FUNCTION "FC_GRP_82" : VOID
TITLE =GROUP =82
{ S7_language := '9(1) Angielski (Stany Zjednoczone)  11.01.2022  09:45:15' }
VERSION : 0.1


VAR_TEMP
  CL : "UDT_CABINET";	//CABINET LOCAL
  CR : "UDT_CABINET";	//CABINET REMOTE
  RelError : BOOL ;	//ERROR RELEASE
  RelErrorCL : BOOL ;	//ERROR RELEASE FROM CABINET LOCAL
  RelErrorCR : BOOL ;	//ERROR RELEASE FROM CABINET REMOTE
  RelControl : BOOL ;	//CONTROL RELEASE
  RelControlCL : BOOL ;	//CONTROL RELEASE FROM CABINET LOCAL
  RelControlCR : BOOL ;	//CONTROL RELEASE FROM CABINET REMOTE
  ErrorConfirm : BOOL ;	//ERROR CONFIRM
  AutoOn : BOOL ;	//AUTOMATIC ON
  AutoOff : BOOL ;	//AUTOMATIC OFF
  LAMP_ON : BOOL ;
  Setpoint_82FAN91_reached : BOOL ;
  Setpoint_82FAN91_div : BOOL ;
  Setpoint_82FAN92_reached : BOOL ;
  Setpoint_82FAN92_div : BOOL ;
END_VAR
BEGIN
NETWORK
TITLE =GLOBAL SIGNALS
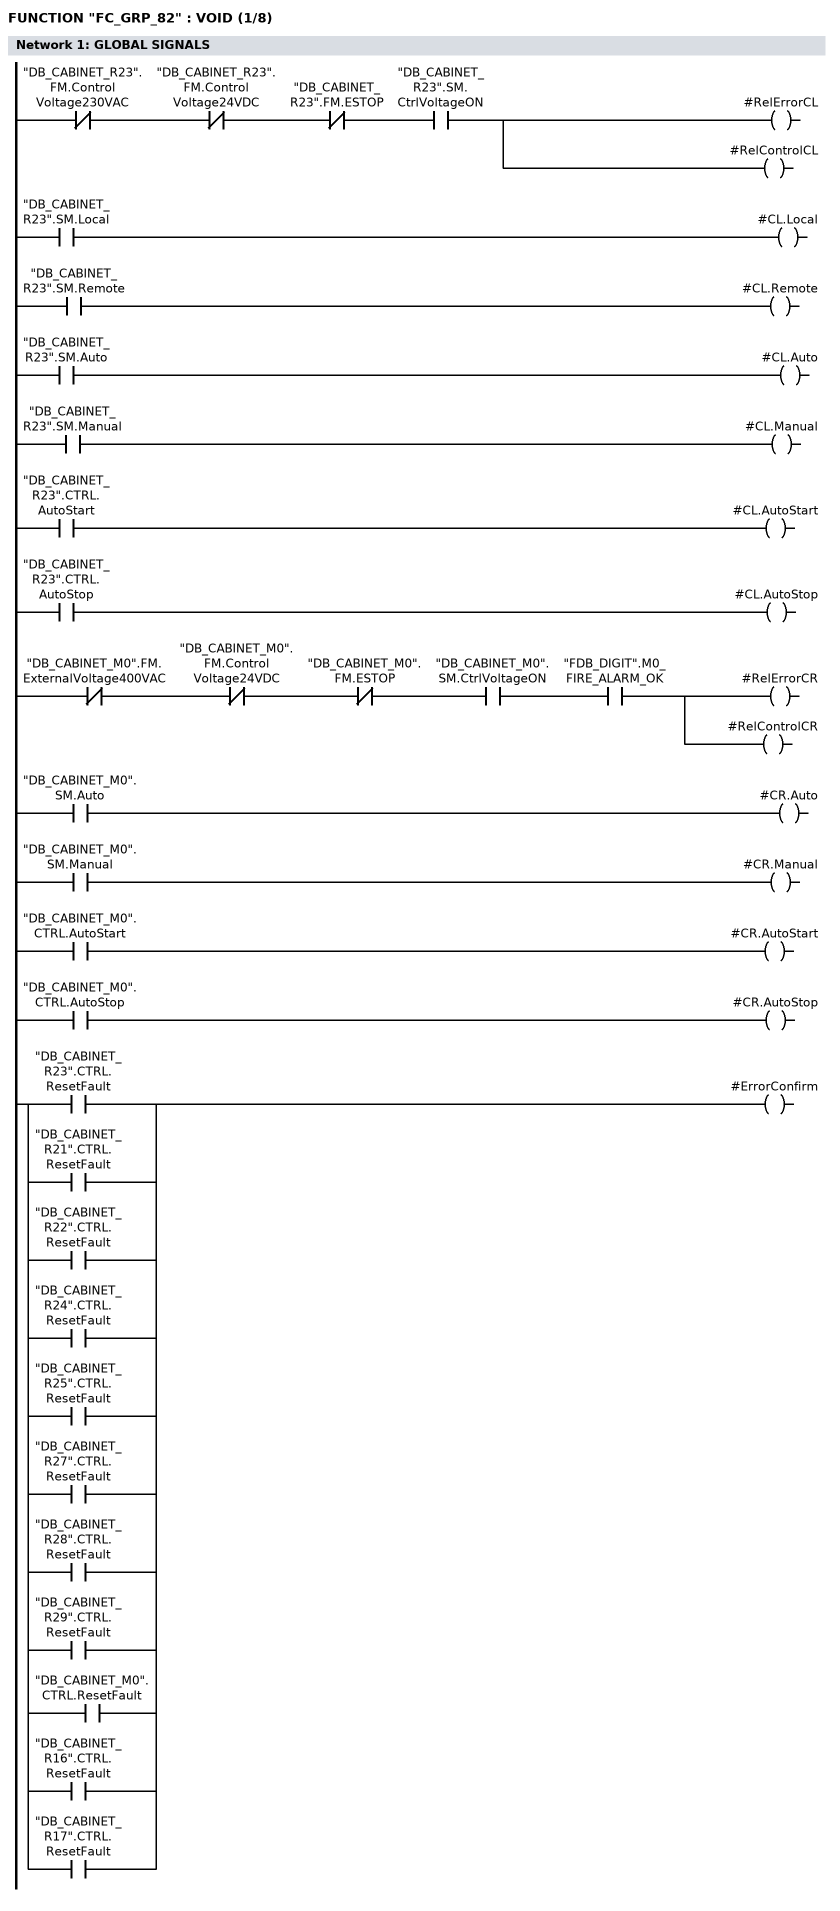
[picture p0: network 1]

// LOCAL
      UN    "DB_CABINET_R23".FM.ControlVoltage230VAC;
      UN    "DB_CABINET_R23".FM.ControlVoltage24VDC;
//      UN    "DB_CABINET_R23".FM.ControlVoltage230VAC_MS
      UN    "DB_CABINET_R23".FM.ESTOP;
      U     "DB_CABINET_R23".SM.CtrlVoltageON;
      =     #RelErrorCL;
      =     #RelControlCL;

      U     "DB_CABINET_R23".SM.Local;
      =     #CL.Local;
      U     "DB_CABINET_R23".SM.Remote;
      =     #CL.Remote;
      U     "DB_CABINET_R23".SM.Auto;
      =     #CL.Auto;
      U     "DB_CABINET_R23".SM.Manual;
      =     #CL.Manual;
      U     "DB_CABINET_R23".CTRL.AutoStart;
      =     #CL.AutoStart;
      U     "DB_CABINET_R23".CTRL.AutoStop;
      =     #CL.AutoStop;

// REMOTE
      UN    "DB_CABINET_M0".FM.ExternalVoltage400VAC;
      UN    "DB_CABINET_M0".FM.ControlVoltage24VDC;
//      UN    "DB_CABINET_M0".FM.ControlVoltage230VAC_MS
      UN    "DB_CABINET_M0".FM.ESTOP;
      U     "DB_CABINET_M0".SM.CtrlVoltageON;
      U     "FDB_DIGIT".M0_FIRE_ALARM_OK;
      =     #RelErrorCR;
      =     #RelControlCR;

      U     "DB_CABINET_M0".SM.Auto;
      =     #CR.Auto;
      U     "DB_CABINET_M0".SM.Manual;
      =     #CR.Manual;
      U     "DB_CABINET_M0".CTRL.AutoStart;
      =     #CR.AutoStart;
      U     "DB_CABINET_M0".CTRL.AutoStop;
      =     #CR.AutoStop;

      U     "DB_CABINET_R23".CTRL.ResetFault;
      O     "DB_CABINET_R21".CTRL.ResetFault;
      O     "DB_CABINET_R22".CTRL.ResetFault;
      O     "DB_CABINET_R24".CTRL.ResetFault;
      O     "DB_CABINET_R25".CTRL.ResetFault;
      O     "DB_CABINET_R27".CTRL.ResetFault;
      O     "DB_CABINET_R28".CTRL.ResetFault;
      O     "DB_CABINET_R29".CTRL.ResetFault;
      O     "DB_CABINET_M0".CTRL.ResetFault;
      O     "DB_CABINET_R16".CTRL.ResetFault;
      O     "DB_CABINET_R17".CTRL.ResetFault;
      =     #ErrorConfirm;

NETWORK
TITLE ==82FTR20-B33 FILTER PRESSURE MONITORING
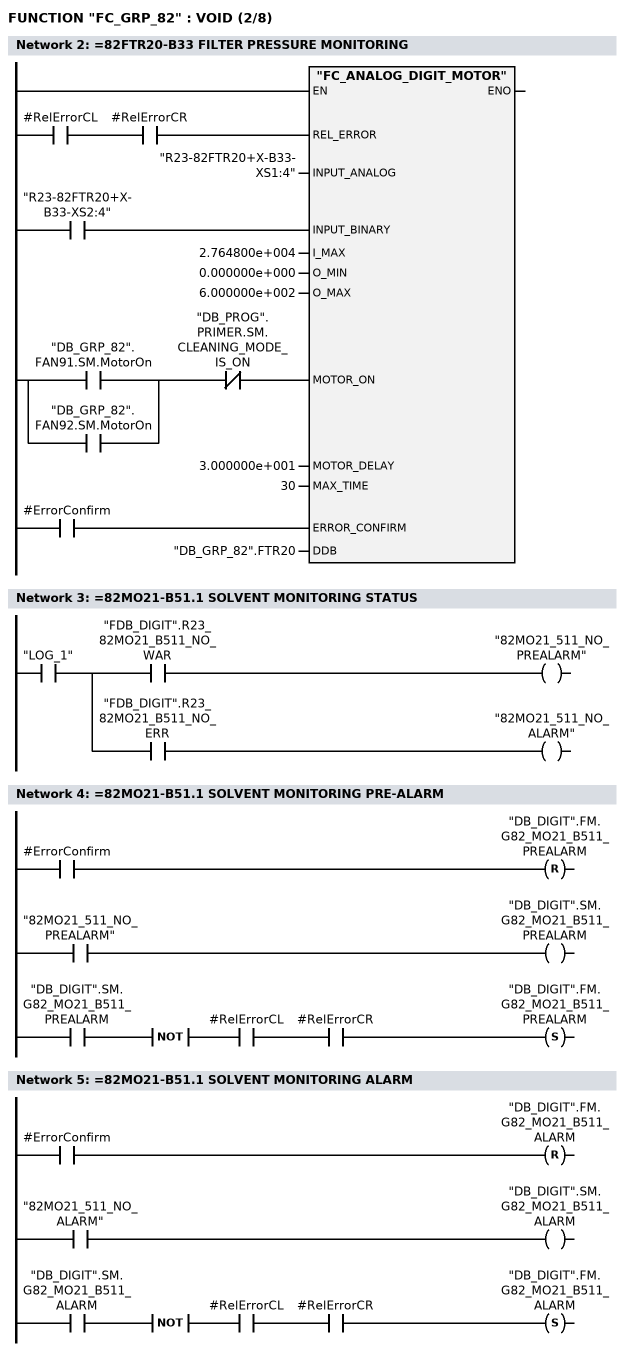
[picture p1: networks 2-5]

      U     #RelErrorCL;
      U     #RelErrorCR;
      =     L      6.0;
      BLD   103;
      U     "R23-82FTR20+X-B33-XS2:4";
      =     L      6.1;
      BLD   103;
      U(    ;
      O     "DB_GRP_82".FAN91.SM.MotorOn;
      O     "DB_GRP_82".FAN92.SM.MotorOn;
      )     ;
      UN    "DB_PROG".PRIMER.SM.CLEANING_MODE_IS_ON;
      =     L      6.2;
      BLD   103;
      U     #ErrorConfirm;
      =     L      6.3;
      BLD   103;
      CALL "FC_ANALOG_DIGIT_MOTOR" (
           REL_ERROR                := L      6.0,
           INPUT_ANALOG             := "R23-82FTR20+X-B33-XS1:4",
           INPUT_BINARY             := L      6.1,
           I_MAX                    := 2.764800e+004,
           O_MIN                    := 0.000000e+000,
           O_MAX                    := 6.000000e+002,
           MOTOR_ON                 := L      6.2,
           MOTOR_DELAY              := 3.000000e+001,
           MAX_TIME                 := 30,
           ERROR_CONFIRM            := L      6.3,
           DDB                      := "DB_GRP_82".FTR20);
      NOP   0;
NETWORK
TITLE ==82MO21-B51.1 SOLVENT MONITORING STATUS

      U     "LOG_1";
      =     L      6.0;
      U     L      6.0;
      U     "FDB_DIGIT".R23_82MO21_B511_NO_WAR;
      =     "82MO21_511_NO_PREALARM";
      U     L      6.0;
      U     "FDB_DIGIT".R23_82MO21_B511_NO_ERR;
      =     "82MO21_511_NO_ALARM";
NETWORK
TITLE ==82MO21-B51.1 SOLVENT MONITORING PRE-ALARM

      U     #ErrorConfirm;
      R     "DB_DIGIT".FM.G82_MO21_B511_PREALARM;
      U     "82MO21_511_NO_PREALARM";
      =     "DB_DIGIT".SM.G82_MO21_B511_PREALARM;
      U     "DB_DIGIT".SM.G82_MO21_B511_PREALARM;
      NOT   ;
      U     #RelErrorCL;
      U     #RelErrorCR;
      S     "DB_DIGIT".FM.G82_MO21_B511_PREALARM;
      NOP   0;
NETWORK
TITLE ==82MO21-B51.1 SOLVENT MONITORING ALARM

      U     #ErrorConfirm;
      R     "DB_DIGIT".FM.G82_MO21_B511_ALARM;
      U     "82MO21_511_NO_ALARM";
      =     "DB_DIGIT".SM.G82_MO21_B511_ALARM;
      U     "DB_DIGIT".SM.G82_MO21_B511_ALARM;
      NOT   ;
      U     #RelErrorCL;
      U     #RelErrorCR;
      S     "DB_DIGIT".FM.G82_MO21_B511_ALARM;
      NOP   0;
NETWORK
TITLE ==82MO21-B51.1 SOLVENT MONITORING ANALOG
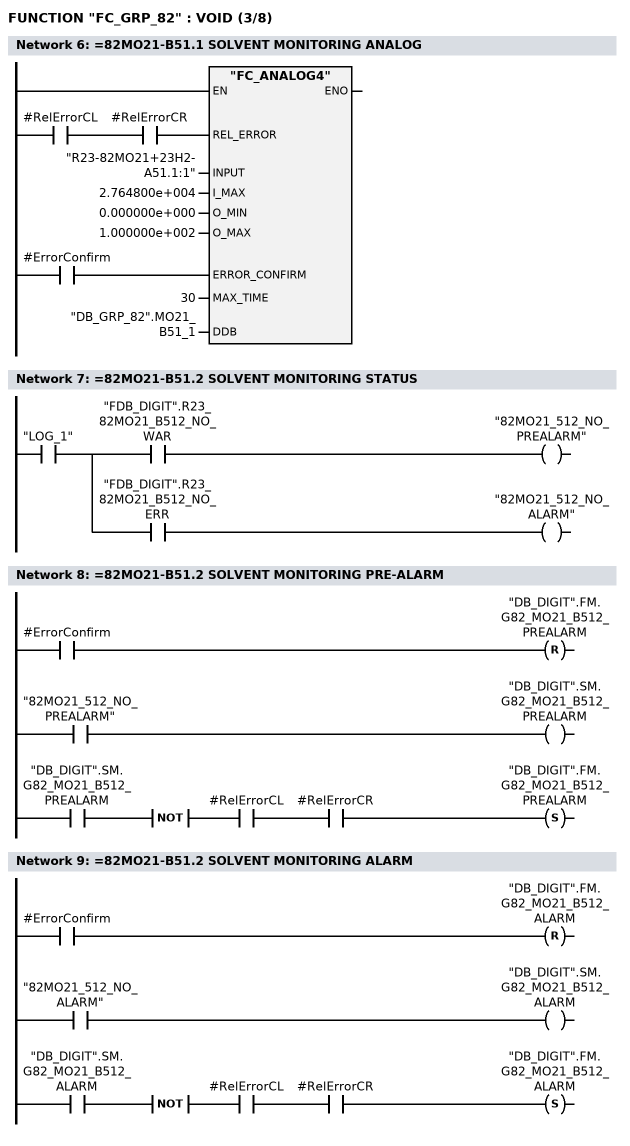
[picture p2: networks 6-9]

      U     #RelErrorCL;
      U     #RelErrorCR;
      =     L      6.0;
      BLD   103;
      U     #ErrorConfirm;
      =     L      6.1;
      BLD   103;
      CALL "FC_ANALOG4" (
           REL_ERROR                := L      6.0,
           INPUT                    := "R23-82MO21+23H2-A51.1:1",
           I_MAX                    := 2.764800e+004,
           O_MIN                    := 0.000000e+000,
           O_MAX                    := 1.000000e+002,
           ERROR_CONFIRM            := L      6.1,
           MAX_TIME                 := 30,
           DDB                      := "DB_GRP_82".MO21_B51_1);
      NOP   0;
NETWORK
TITLE ==82MO21-B51.2 SOLVENT MONITORING STATUS

      U     "LOG_1";
      =     L      6.0;
      U     L      6.0;
      U     "FDB_DIGIT".R23_82MO21_B512_NO_WAR;
      =     "82MO21_512_NO_PREALARM";
      U     L      6.0;
      U     "FDB_DIGIT".R23_82MO21_B512_NO_ERR;
      =     "82MO21_512_NO_ALARM";
NETWORK
TITLE ==82MO21-B51.2 SOLVENT MONITORING PRE-ALARM

      U     #ErrorConfirm;
      R     "DB_DIGIT".FM.G82_MO21_B512_PREALARM;
      U     "82MO21_512_NO_PREALARM";
      =     "DB_DIGIT".SM.G82_MO21_B512_PREALARM;
      U     "DB_DIGIT".SM.G82_MO21_B512_PREALARM;
      NOT   ;
      U     #RelErrorCL;
      U     #RelErrorCR;
      S     "DB_DIGIT".FM.G82_MO21_B512_PREALARM;
      NOP   0;
NETWORK
TITLE ==82MO21-B51.2 SOLVENT MONITORING ALARM

      U     #ErrorConfirm;
      R     "DB_DIGIT".FM.G82_MO21_B512_ALARM;
      U     "82MO21_512_NO_ALARM";
      =     "DB_DIGIT".SM.G82_MO21_B512_ALARM;
      U     "DB_DIGIT".SM.G82_MO21_B512_ALARM;
      NOT   ;
      U     #RelErrorCL;
      U     #RelErrorCR;
      S     "DB_DIGIT".FM.G82_MO21_B512_ALARM;
      NOP   0;
NETWORK
TITLE ==82MO21-B51.2 SOLVENT MONITORING ANALOG
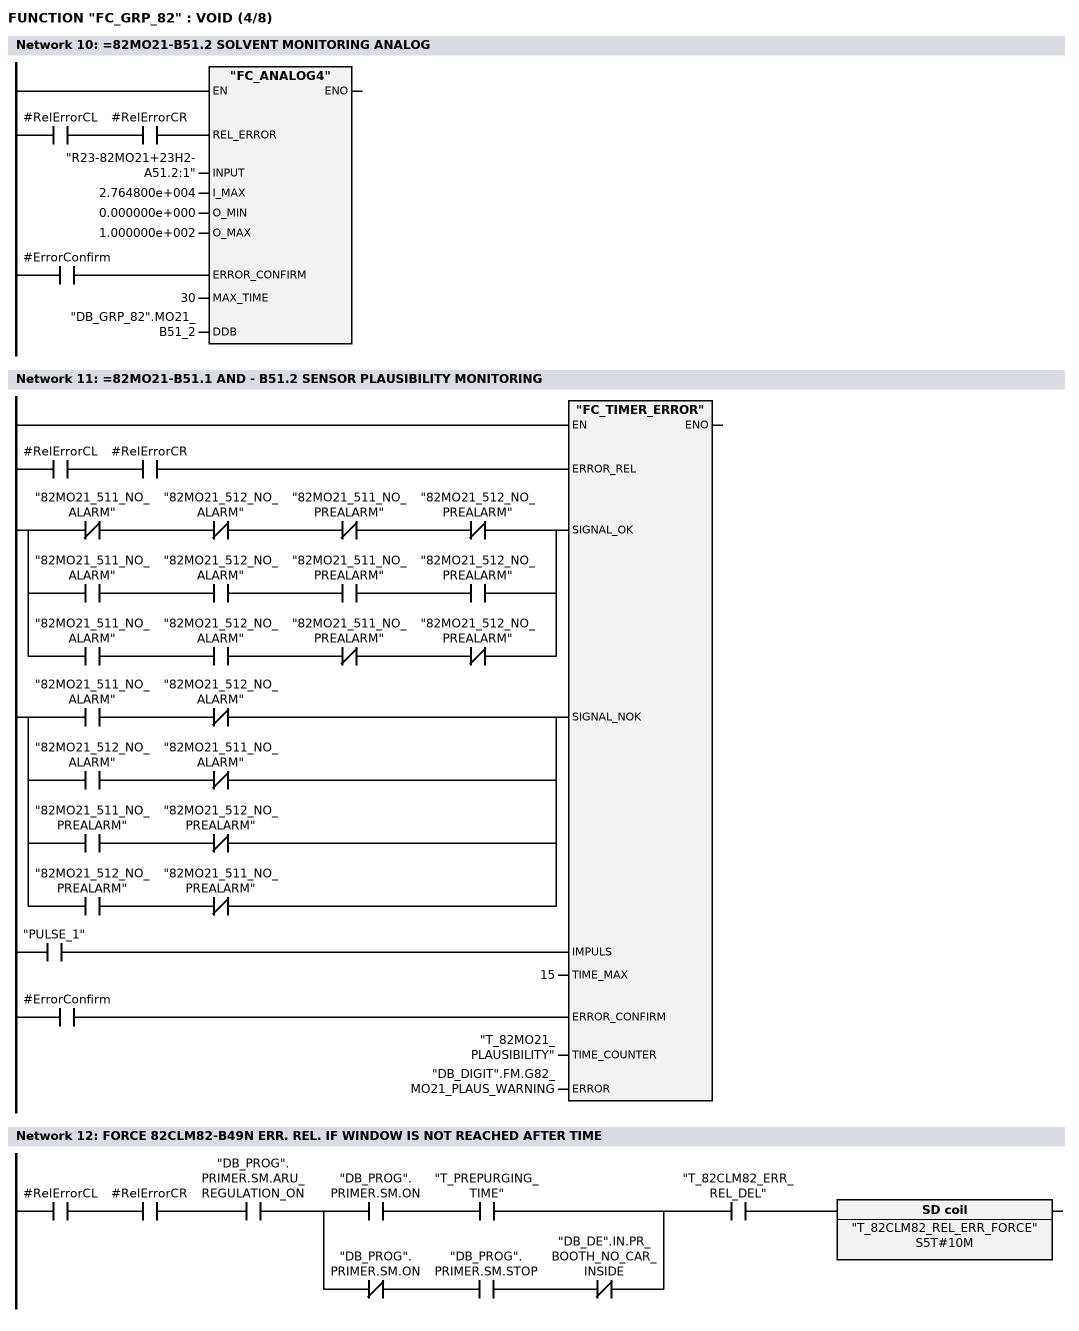
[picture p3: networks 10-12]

      U     #RelErrorCL;
      U     #RelErrorCR;
      =     L      6.0;
      BLD   103;
      U     #ErrorConfirm;
      =     L      6.1;
      BLD   103;
      CALL "FC_ANALOG4" (
           REL_ERROR                := L      6.0,
           INPUT                    := "R23-82MO21+23H2-A51.2:1",
           I_MAX                    := 2.764800e+004,
           O_MIN                    := 0.000000e+000,
           O_MAX                    := 1.000000e+002,
           ERROR_CONFIRM            := L      6.1,
           MAX_TIME                 := 30,
           DDB                      := "DB_GRP_82".MO21_B51_2);
      NOP   0;
NETWORK
TITLE ==82MO21-B51.1 AND - B51.2 SENSOR PLAUSIBILITY MONITORING

      U     #RelErrorCL;
      U     #RelErrorCR;
      =     L      6.0;
      BLD   103;
      U(    ;
      UN    "82MO21_511_NO_ALARM";
      UN    "82MO21_512_NO_ALARM";
      UN    "82MO21_511_NO_PREALARM";
      UN    "82MO21_512_NO_PREALARM";
      O     ;
      U     "82MO21_511_NO_ALARM";
      U     "82MO21_512_NO_ALARM";
      U     "82MO21_511_NO_PREALARM";
      U     "82MO21_512_NO_PREALARM";
      O     ;
      U     "82MO21_511_NO_ALARM";
      U     "82MO21_512_NO_ALARM";
      UN    "82MO21_511_NO_PREALARM";
      UN    "82MO21_512_NO_PREALARM";
      )     ;
      =     L      6.1;
      BLD   103;
      U(    ;
      U     "82MO21_511_NO_ALARM";
      UN    "82MO21_512_NO_ALARM";
      O     ;
      U     "82MO21_512_NO_ALARM";
      UN    "82MO21_511_NO_ALARM";
      O     ;
      U     "82MO21_511_NO_PREALARM";
      UN    "82MO21_512_NO_PREALARM";
      O     ;
      U     "82MO21_512_NO_PREALARM";
      UN    "82MO21_511_NO_PREALARM";
      )     ;
      =     L      6.2;
      BLD   103;
      U     "PULSE_1";
      =     L      6.3;
      BLD   103;
      U     #ErrorConfirm;
      =     L      6.4;
      BLD   103;
      CALL "FC_TIMER_ERROR" (
           ERROR_REL                := L      6.0,
           SIGNAL_OK                := L      6.1,
           SIGNAL_NOK               := L      6.2,
           IMPULS                   := L      6.3,
           TIME_MAX                 := 15,
           ERROR_CONFIRM            := L      6.4,
           TIME_COUNTER             := "T_82MO21_PLAUSIBILITY",
           ERROR                    := "DB_DIGIT".FM.G82_MO21_PLAUS_WARNING);
      NOP   0;
NETWORK
TITLE =FORCE 82CLM82-B49N ERR. REL. IF WINDOW IS NOT REACHED AFTER TIME

      U     #RelErrorCL;
      U     #RelErrorCR;
      U     "DB_PROG".PRIMER.SM.ARU_REGULATION_ON;
      U(    ;
      U     "DB_PROG".PRIMER.SM.ON;
      U     "T_PREPURGING_TIME";
      O     ;
      UN    "DB_PROG".PRIMER.SM.ON;
      U     "DB_PROG".PRIMER.SM.STOP;
      UN    "DB_DE".IN.PR_BOOTH_NO_CAR_INSIDE;
      )     ;
      U     "T_82CLM82_ERR_REL_DEL";
      L     S5T#10M;
      SE    "T_82CLM82_REL_ERR_FORCE";
      NOP   0;
      NOP   0;
      NOP   0;
      NOP   0;
NETWORK
TITLE ==82CLM82-B49N SETPOINT CHANGED
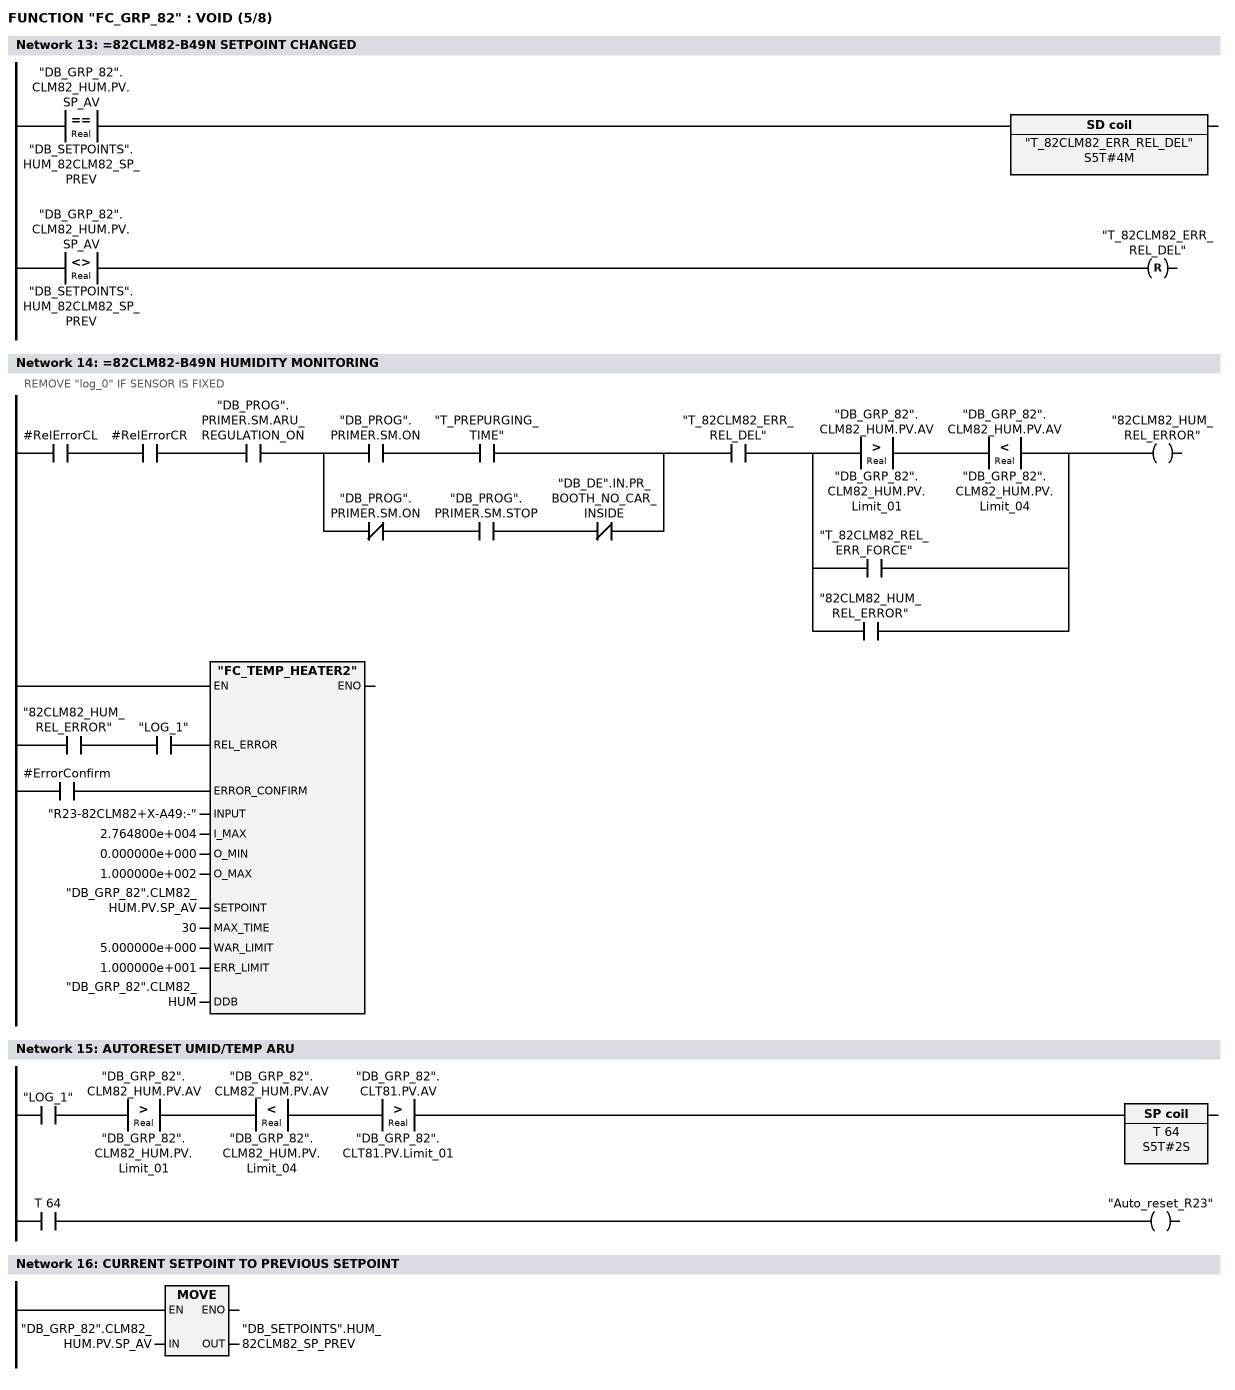
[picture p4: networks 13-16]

      U(    ;
      L     "DB_GRP_82".CLM82_HUM.PV.SP_AV;
      L     "DB_SETPOINTS".HUM_82CLM82_SP_PREV;
      ==R   ;
      )     ;
      L     S5T#4M;
      SE    "T_82CLM82_ERR_REL_DEL";
      U(    ;
      L     "DB_GRP_82".CLM82_HUM.PV.SP_AV;
      L     "DB_SETPOINTS".HUM_82CLM82_SP_PREV;
      <>R   ;
      )     ;
      R     "T_82CLM82_ERR_REL_DEL";
      NOP   0;
      NOP   0;
      NOP   0;
NETWORK
TITLE ==82CLM82-B49N HUMIDITY MONITORING
//
//
//
//
//
//
//
//
//
//REMOVE "log_0" IF SENSOR IS FIXED
      U     #RelErrorCL;
      U     #RelErrorCR;
      U     "DB_PROG".PRIMER.SM.ARU_REGULATION_ON;
      U(    ;
      U     "DB_PROG".PRIMER.SM.ON;
      U     "T_PREPURGING_TIME";
      O     ;
      UN    "DB_PROG".PRIMER.SM.ON;
      U     "DB_PROG".PRIMER.SM.STOP;
      UN    "DB_DE".IN.PR_BOOTH_NO_CAR_INSIDE;
      )     ;
      U     "T_82CLM82_ERR_REL_DEL";
      U(    ;
      U(    ;
      L     "DB_GRP_82".CLM82_HUM.PV.AV;
      L     "DB_GRP_82".CLM82_HUM.PV.Limit_01;
      >R    ;
      )     ;
      U(    ;
      L     "DB_GRP_82".CLM82_HUM.PV.AV;
      L     "DB_GRP_82".CLM82_HUM.PV.Limit_04;
      <R    ;
      )     ;
      O     "T_82CLM82_REL_ERR_FORCE";
      O     "82CLM82_HUM_REL_ERROR";
      )     ;
      =     "82CLM82_HUM_REL_ERROR";
      U     "82CLM82_HUM_REL_ERROR";
      U     "LOG_1";
      =     L      6.0;
      BLD   103;
      U     #ErrorConfirm;
      =     L      6.1;
      BLD   103;
      CALL "FC_TEMP_HEATER2" (
           REL_ERROR                := L      6.0,
           ERROR_CONFIRM            := L      6.1,
           INPUT                    := "R23-82CLM82+X-A49:-",
           I_MAX                    := 2.764800e+004,
           O_MIN                    := 0.000000e+000,
           O_MAX                    := 1.000000e+002,
           SETPOINT                 := "DB_GRP_82".CLM82_HUM.PV.SP_AV,
           MAX_TIME                 := 30,
           WAR_LIMIT                := 5.000000e+000,
           ERR_LIMIT                := 1.000000e+001,
           DDB                      := "DB_GRP_82".CLM82_HUM);
      NOP   0;
NETWORK
TITLE =AUTORESET UMID/TEMP ARU

      U     "LOG_1";
      U(    ;
      L     "DB_GRP_82".CLM82_HUM.PV.AV;
      L     "DB_GRP_82".CLM82_HUM.PV.Limit_01;
      >R    ;
      )     ;
      U(    ;
      L     "DB_GRP_82".CLM82_HUM.PV.AV;
      L     "DB_GRP_82".CLM82_HUM.PV.Limit_04;
      <R    ;
      )     ;
      U(    ;
      L     "DB_GRP_82".CLT81.PV.AV;
      L     "DB_GRP_82".CLT81.PV.Limit_01;
      >R    ;
      )     ;
      L     S5T#2S;
      SI    T     64;
      NOP   0;
      NOP   0;
      NOP   0;
      U     T     64;
      =     "Auto_reset_R23";
NETWORK
TITLE =CURRENT SETPOINT TO PREVIOUS SETPOINT

      L     "DB_GRP_82".CLM82_HUM.PV.SP_AV;
      T     "DB_SETPOINTS".HUM_82CLM82_SP_PREV;
      NOP   0;
NETWORK
TITLE =FORCE 82CLT81-B40N ERR. REL. IF WINDOW IS NOT REACHED AFTER TIME
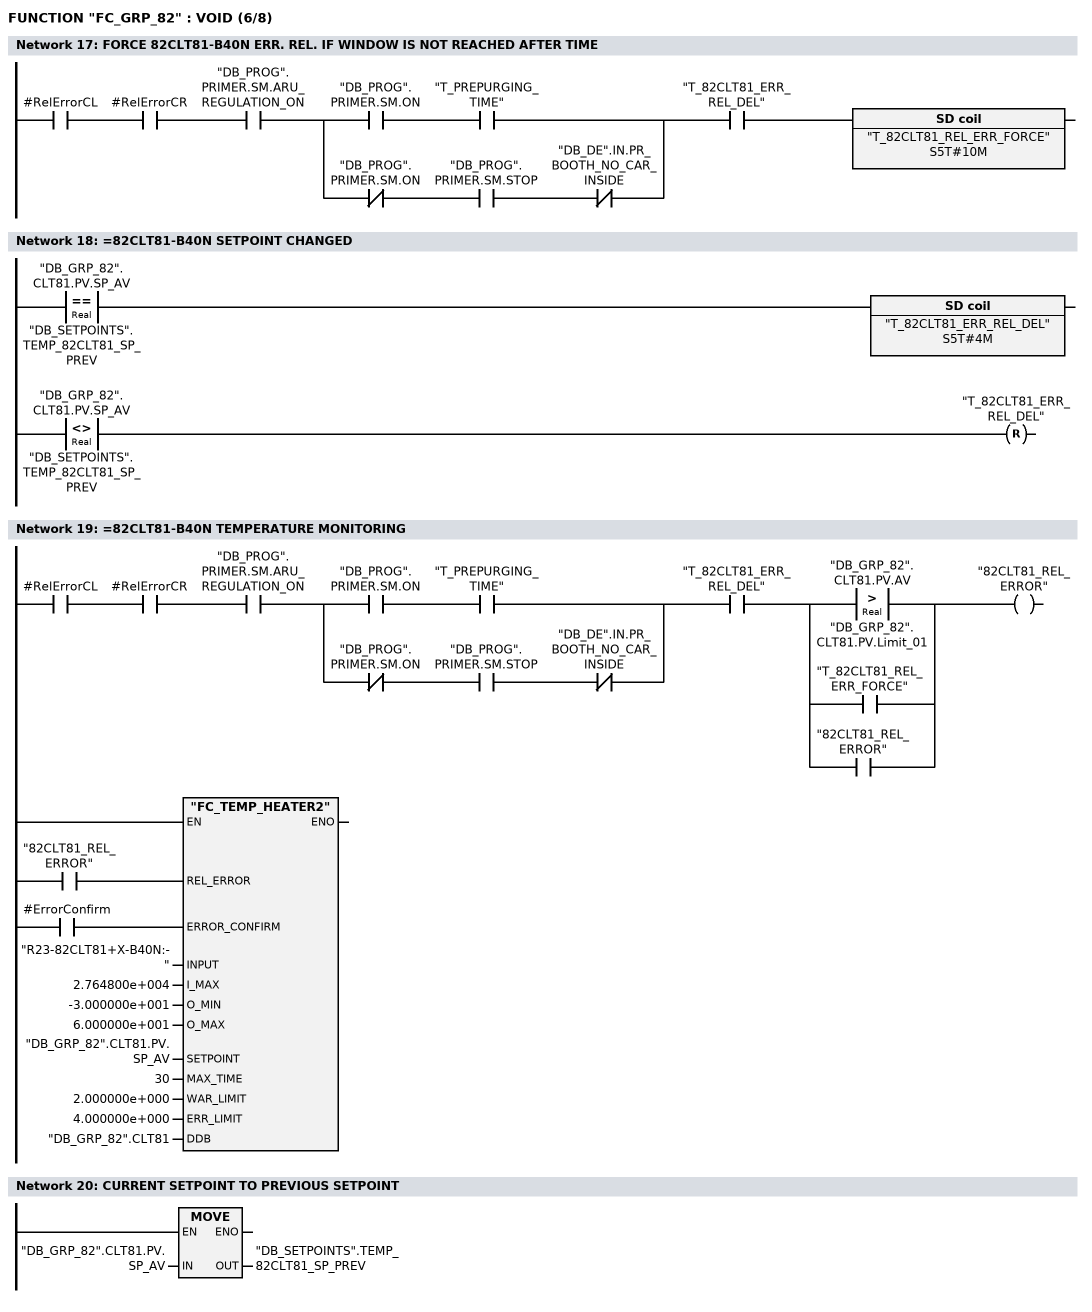
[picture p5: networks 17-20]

      U     #RelErrorCL;
      U     #RelErrorCR;
      U     "DB_PROG".PRIMER.SM.ARU_REGULATION_ON;
      U(    ;
      U     "DB_PROG".PRIMER.SM.ON;
      U     "T_PREPURGING_TIME";
      O     ;
      UN    "DB_PROG".PRIMER.SM.ON;
      U     "DB_PROG".PRIMER.SM.STOP;
      UN    "DB_DE".IN.PR_BOOTH_NO_CAR_INSIDE;
      )     ;
      U     "T_82CLT81_ERR_REL_DEL";
      L     S5T#10M;
      SE    "T_82CLT81_REL_ERR_FORCE";
      NOP   0;
      NOP   0;
      NOP   0;
      NOP   0;
NETWORK
TITLE ==82CLT81-B40N SETPOINT CHANGED

      U(    ;
      L     "DB_GRP_82".CLT81.PV.SP_AV;
      L     "DB_SETPOINTS".TEMP_82CLT81_SP_PREV;
      ==R   ;
      )     ;
      L     S5T#4M;
      SE    "T_82CLT81_ERR_REL_DEL";
      U(    ;
      L     "DB_GRP_82".CLT81.PV.SP_AV;
      L     "DB_SETPOINTS".TEMP_82CLT81_SP_PREV;
      <>R   ;
      )     ;
      R     "T_82CLT81_ERR_REL_DEL";
      NOP   0;
      NOP   0;
      NOP   0;
NETWORK
TITLE ==82CLT81-B40N TEMPERATURE MONITORING

      U     #RelErrorCL;
      U     #RelErrorCR;
      U     "DB_PROG".PRIMER.SM.ARU_REGULATION_ON;
      U(    ;
      U     "DB_PROG".PRIMER.SM.ON;
      U     "T_PREPURGING_TIME";
      O     ;
      UN    "DB_PROG".PRIMER.SM.ON;
      U     "DB_PROG".PRIMER.SM.STOP;
      UN    "DB_DE".IN.PR_BOOTH_NO_CAR_INSIDE;
      )     ;
      U     "T_82CLT81_ERR_REL_DEL";
      U(    ;
      O(    ;
      L     "DB_GRP_82".CLT81.PV.AV;
      L     "DB_GRP_82".CLT81.PV.Limit_01;
      >R    ;
      )     ;
      O     "T_82CLT81_REL_ERR_FORCE";
      O     "82CLT81_REL_ERROR";
      )     ;
      =     "82CLT81_REL_ERROR";
      U     "82CLT81_REL_ERROR";
      =     L      6.0;
      BLD   103;
      U     #ErrorConfirm;
      =     L      6.1;
      BLD   103;
      CALL "FC_TEMP_HEATER2" (
           REL_ERROR                := L      6.0,
           ERROR_CONFIRM            := L      6.1,
           INPUT                    := "R23-82CLT81+X-B40N:-",
           I_MAX                    := 2.764800e+004,
           O_MIN                    := -3.000000e+001,
           O_MAX                    := 6.000000e+001,
           SETPOINT                 := "DB_GRP_82".CLT81.PV.SP_AV,
           MAX_TIME                 := 30,
           WAR_LIMIT                := 2.000000e+000,
           ERR_LIMIT                := 4.000000e+000,
           DDB                      := "DB_GRP_82".CLT81);
      NOP   0;
NETWORK
TITLE =CURRENT SETPOINT TO PREVIOUS SETPOINT

      L     "DB_GRP_82".CLT81.PV.SP_AV;
      T     "DB_SETPOINTS".TEMP_82CLT81_SP_PREV;
      NOP   0;
NETWORK
TITLE ==82CLM82-B49N TEMPERATURE MONITORING
//IN PAP THERE IS INFORMATION THAT THIS TEMPERATURE SENSOR IS NOT USED (THERE IS
//ONE DEVICE MEASURING HUMIDITY AND TEMPERATURE)
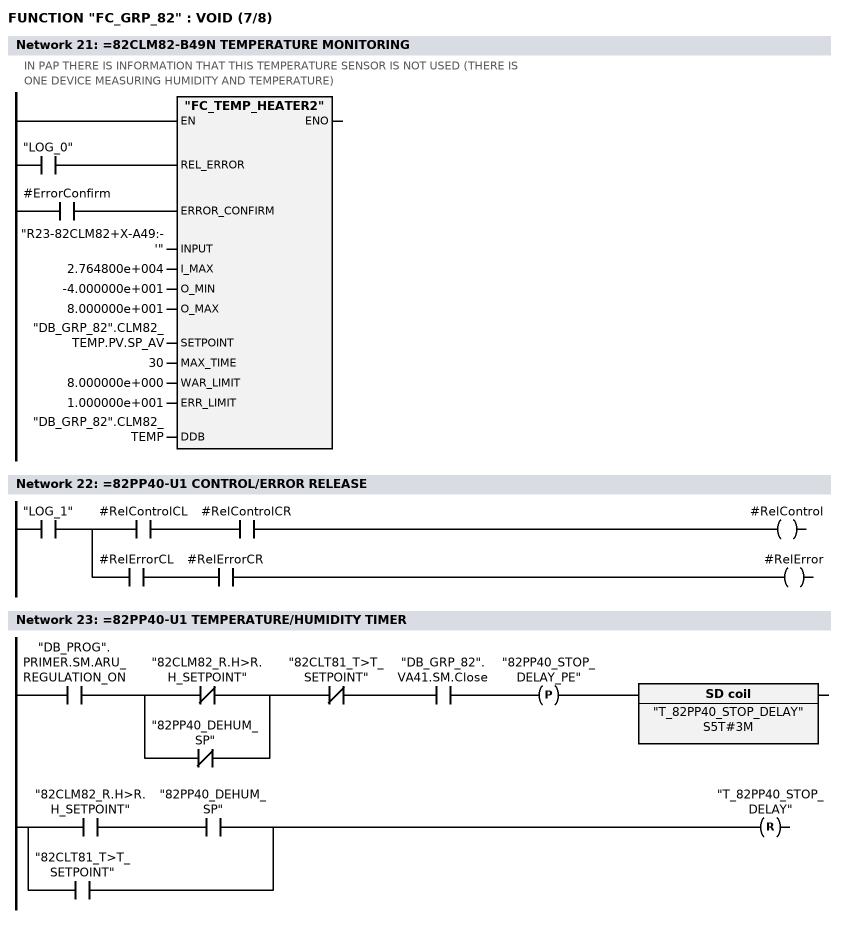
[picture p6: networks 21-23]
      U     "LOG_0";
      =     L      6.0;
      BLD   103;
      U     #ErrorConfirm;
      =     L      6.1;
      BLD   103;
      CALL "FC_TEMP_HEATER2" (
           REL_ERROR                := L      6.0,
           ERROR_CONFIRM            := L      6.1,
           INPUT                    := "R23-82CLM82+X-A49:-'",
           I_MAX                    := 2.764800e+004,
           O_MIN                    := -4.000000e+001,
           O_MAX                    := 8.000000e+001,
           SETPOINT                 := "DB_GRP_82".CLM82_TEMP.PV.SP_AV,
           MAX_TIME                 := 30,
           WAR_LIMIT                := 8.000000e+000,
           ERR_LIMIT                := 1.000000e+001,
           DDB                      := "DB_GRP_82".CLM82_TEMP);
      NOP   0;
NETWORK
TITLE ==82PP40-U1 CONTROL/ERROR RELEASE

      U     "LOG_1";
      =     L      6.0;
      U     L      6.0;
      U     #RelControlCL;
      U     #RelControlCR;
      =     #RelControl;
      U     L      6.0;
      U     #RelErrorCL;
      U     #RelErrorCR;
      =     #RelError;
NETWORK
TITLE ==82PP40-U1 TEMPERATURE/HUMIDITY TIMER

      U     "DB_PROG".PRIMER.SM.ARU_REGULATION_ON;
      U(    ;
      ON    "82CLM82_R.H>R.H_SETPOINT";
      ON    "82PP40_DEHUM_SP";
      )     ;
      UN    "82CLT81_T>T_SETPOINT";
      U     "DB_GRP_82".VA41.SM.Close;
      FP    "82PP40_STOP_DELAY_PE";
      L     S5T#3M;
      SE    "T_82PP40_STOP_DELAY";
      U(    ;
      U     "82CLM82_R.H>R.H_SETPOINT";
      U     "82PP40_DEHUM_SP";
      O     "82CLT81_T>T_SETPOINT";
      )     ;
      R     "T_82PP40_STOP_DELAY";
      NOP   0;
      NOP   0;
      NOP   0;
NETWORK
TITLE ==82PP40-U1 CONTROL SIGNALS
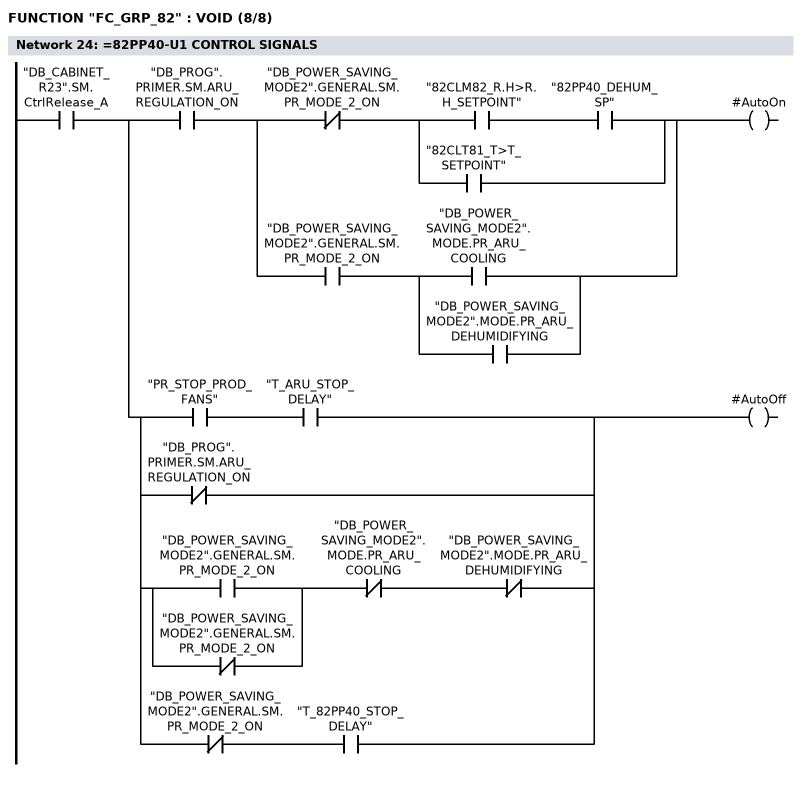
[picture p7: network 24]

      U     "DB_CABINET_R23".SM.CtrlRelease_A;
      =     L      6.0;
      U     L      6.0;
      U     "DB_PROG".PRIMER.SM.ARU_REGULATION_ON;
      U(    ;
      UN    "DB_POWER_SAVING_MODE2".GENERAL.SM.PR_MODE_2_ON;
      U(    ;
      U     "82CLM82_R.H>R.H_SETPOINT";
      U     "82PP40_DEHUM_SP";
      O     "82CLT81_T>T_SETPOINT";
      )     ;
      O     ;
      U     "DB_POWER_SAVING_MODE2".GENERAL.SM.PR_MODE_2_ON;
      U(    ;
      O     "DB_POWER_SAVING_MODE2".MODE.PR_ARU_COOLING;
      O     "DB_POWER_SAVING_MODE2".MODE.PR_ARU_DEHUMIDIFYING;
      )     ;
      )     ;
      =     #AutoOn;
      U     L      6.0;
      U(    ;
      U     "PR_STOP_PROD_FANS";
      U     "T_ARU_STOP_DELAY";
      ON    "DB_PROG".PRIMER.SM.ARU_REGULATION_ON;
      O     ;
      U(    ;
      O     "DB_POWER_SAVING_MODE2".GENERAL.SM.PR_MODE_2_ON;
      ON    "DB_POWER_SAVING_MODE2".GENERAL.SM.PR_MODE_2_ON;
      )     ;
      UN    "DB_POWER_SAVING_MODE2".MODE.PR_ARU_COOLING;
      UN    "DB_POWER_SAVING_MODE2".MODE.PR_ARU_DEHUMIDIFYING;
      O     ;
      UN    "DB_POWER_SAVING_MODE2".GENERAL.SM.PR_MODE_2_ON;
      U     "T_82PP40_STOP_DELAY";
      )     ;
      =     #AutoOff;
NETWORK
TITLE ==82PP40-U1 SETPOINT TRANSFER

      U     "LOG_1";
      =     L      6.0;
      U     L      6.0;
      U     "DB_GRP_82".PP40.SM.AutomaticMode;
      =     L      6.1;
      U     L      6.1;
      UN    "DB_POWER_SAVING_MODE2".GENERAL.SM.PR_MODE_2_ON;
      =     L      6.2;
      U     L      6.2;
      U     "82PP40_DEHUM_SP";
      SPBNB _001;
      L     "DB_SETPOINTS".PUMP_82PP40_DEHUM_SP;
      T     "DB_GRP_82".PP40.PV.SP;
_001: NOP   0;
      U     L      6.2;
      UN    "82PP40_DEHUM_SP";
      SPBNB _002;
      L     "DB_SETPOINTS".PUMP_82PP40_COOL_SP;
      T     "DB_GRP_82".PP40.PV.SP;
_002: NOP   0;
      U     L      6.1;
      U     "DB_POWER_SAVING_MODE2".GENERAL.SM.PR_MODE_2_ON;
      =     L      6.2;
      U     L      6.2;
      U     "DB_POWER_SAVING_MODE2".MODE.PR_ARU_DEHUMIDIFYING;
      SPBNB _003;
      L     "DB_SETPOINTS".PUMP_82PP40_DEHUM_SP;
      T     "DB_GRP_82".PP40.PV.SP;
_003: NOP   0;
      U     L      6.2;
      U     "DB_POWER_SAVING_MODE2".MODE.PR_ARU_COOLING;
      SPBNB _004;
      L     "DB_SETPOINTS".PUMP_82PP40_COOL_SP;
      T     "DB_GRP_82".PP40.PV.SP;
_004: NOP   0;
      U     L      6.0;
      U     "DB_GRP_82".PP40.SM.ManualMode;
      SPBNB _005;
      L     "DB_SETPOINTS".PUMP_82PP40_COOL_SP;
      T     "DB_GRP_82".PP40.PV.SP;
_005: NOP   0;
NETWORK
TITLE ==82PP40-U1 PUMP COLD WATER
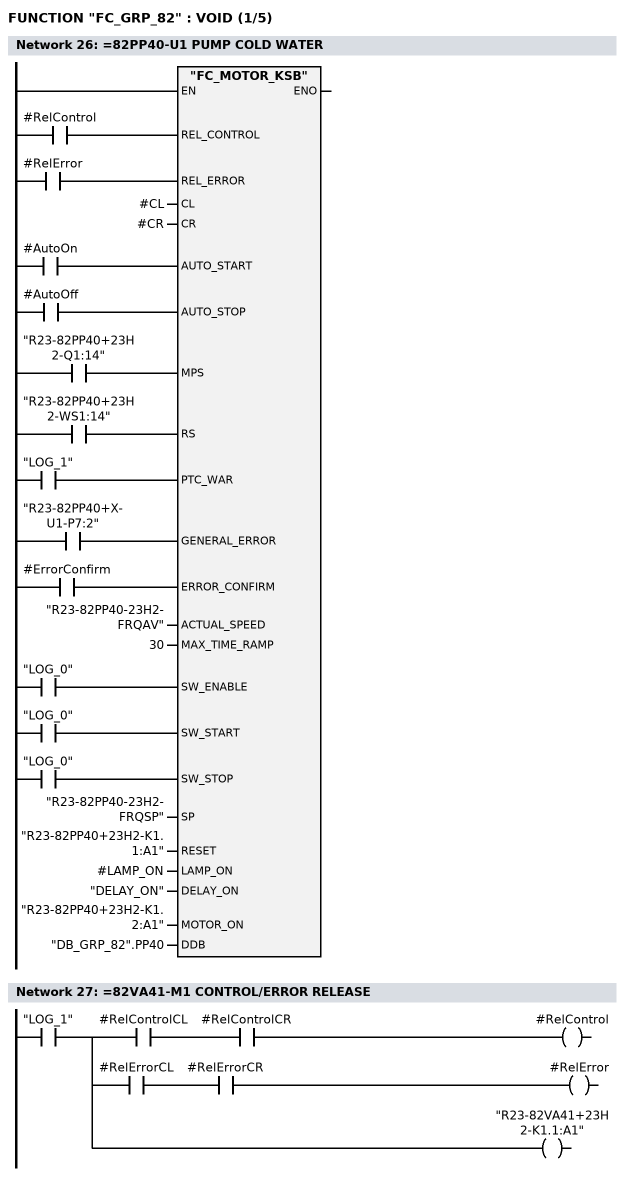
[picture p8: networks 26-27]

      U     #RelControl;
      =     L      6.0;
      BLD   103;
      U     #RelError;
      =     L      6.1;
      BLD   103;
      U     #AutoOn;
      =     L      6.2;
      BLD   103;
      U     #AutoOff;
      =     L      6.3;
      BLD   103;
      U     "R23-82PP40+23H2-Q1:14";
      =     L      6.4;
      BLD   103;
      U     "R23-82PP40+23H2-WS1:14";
      =     L      6.5;
      BLD   103;
      U     "LOG_1";
      =     L      6.6;
      BLD   103;
      U     "R23-82PP40+X-U1-P7:2";
      =     L      6.7;
      BLD   103;
      U     #ErrorConfirm;
      =     L      7.0;
      BLD   103;
      U     "LOG_0";
      =     L      7.1;
      BLD   103;
      U     "LOG_0";
      =     L      7.2;
      BLD   103;
      U     "LOG_0";
      =     L      7.3;
      BLD   103;
      CALL "FC_MOTOR_KSB" (
           REL_CONTROL              := L      6.0,
           REL_ERROR                := L      6.1,
           CL                       := #CL,
           CR                       := #CR,
           AUTO_START               := L      6.2,
           AUTO_STOP                := L      6.3,
           MPS                      := L      6.4,
           RS                       := L      6.5,
           PTC_WAR                  := L      6.6,
           GENERAL_ERROR            := L      6.7,
           ERROR_CONFIRM            := L      7.0,
           ACTUAL_SPEED             := "R23-82PP40-23H2-FRQAV",
           MAX_TIME_RAMP            := 30,
           SW_ENABLE                := L      7.1,
           SW_START                 := L      7.2,
           SW_STOP                  := L      7.3,
           SP                       := "R23-82PP40-23H2-FRQSP",
           RESET                    := "R23-82PP40+23H2-K1.1:A1",
           LAMP_ON                  := #LAMP_ON,
           DELAY_ON                 := "DELAY_ON",
           MOTOR_ON                 := "R23-82PP40+23H2-K1.2:A1",
           DDB                      := "DB_GRP_82".PP40);
      NOP   0;
NETWORK
TITLE ==82VA41-M1 CONTROL/ERROR RELEASE

      U     "LOG_1";
      =     L      6.0;
      U     L      6.0;
      U     #RelControlCL;
      U     #RelControlCR;
      =     #RelControl;
      U     L      6.0;
      U     #RelErrorCL;
      U     #RelErrorCR;
      =     #RelError;
      U     L      6.0;
      BLD   102;
      =     "R23-82VA41+23H2-K1.1:A1";
NETWORK
TITLE ==82VA41-M1 CONTROL VALVE HEATING CONTROL SIGNALS
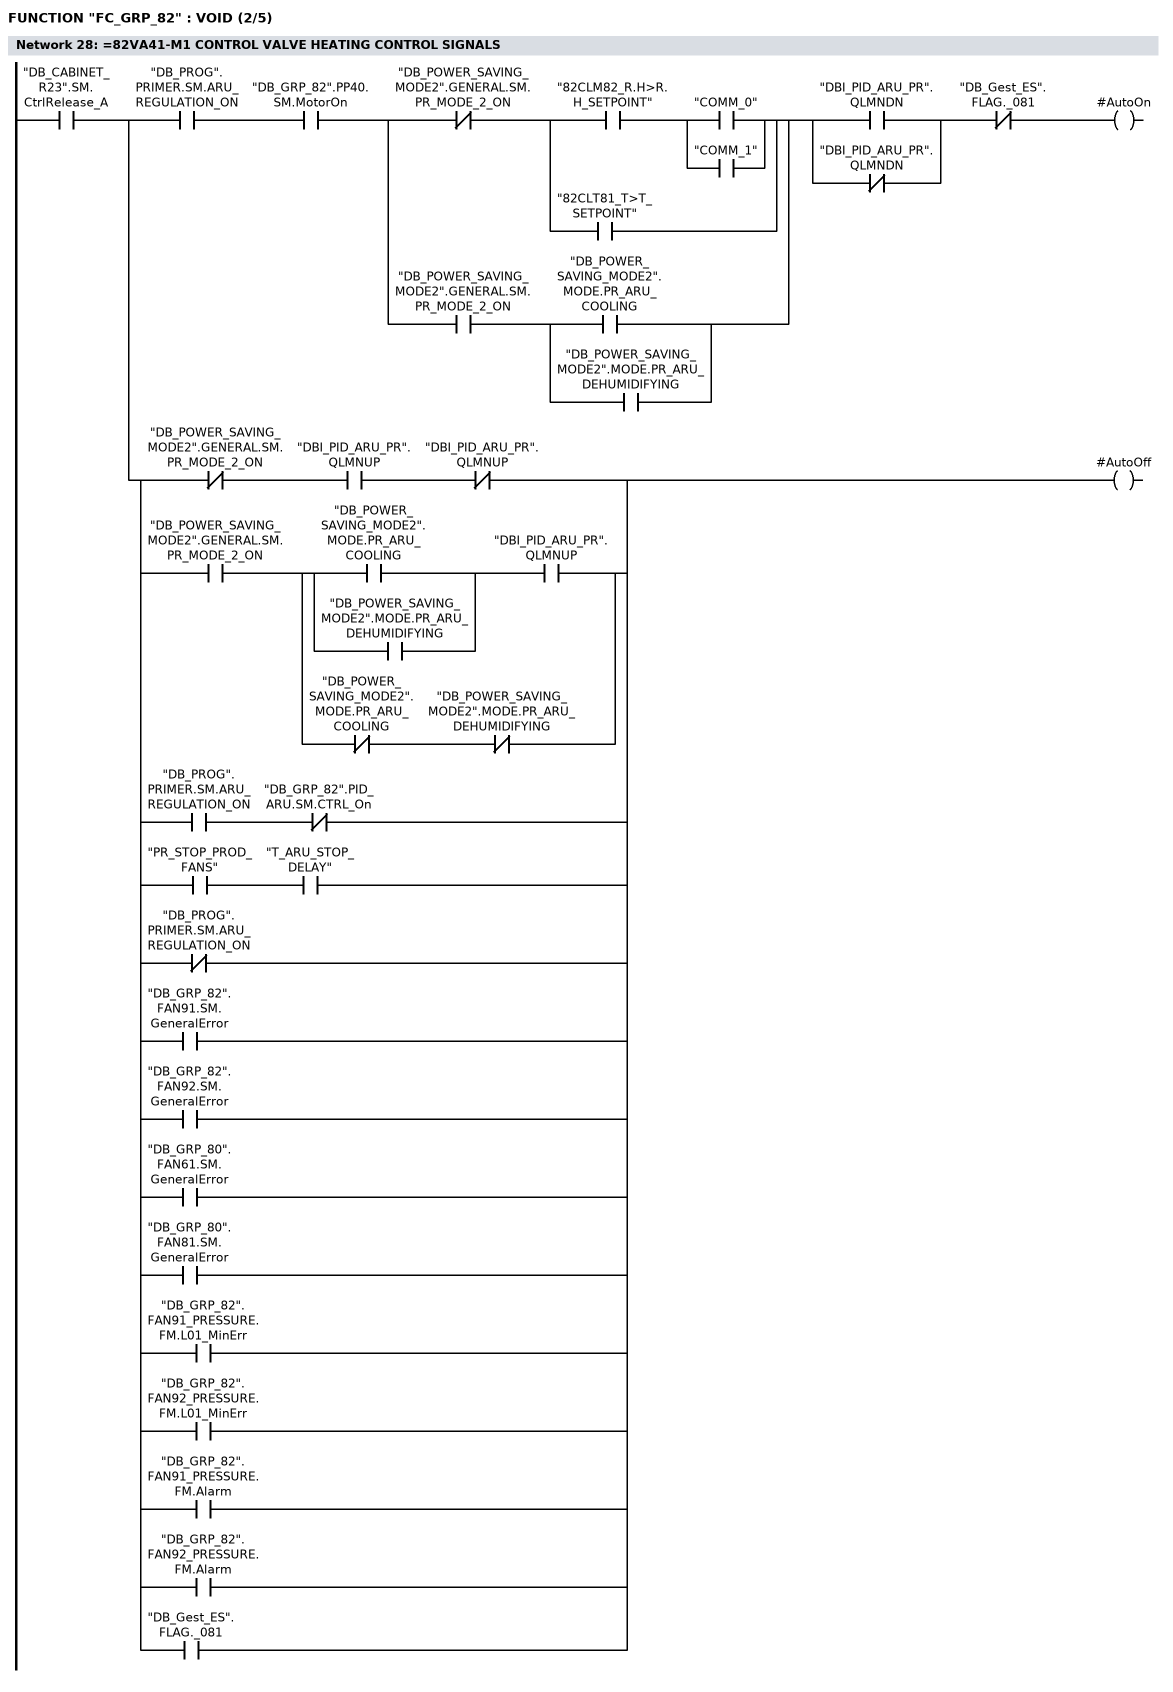
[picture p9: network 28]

      U     "DB_CABINET_R23".SM.CtrlRelease_A;
      =     L      6.0;
      U     L      6.0;
      U     "DB_PROG".PRIMER.SM.ARU_REGULATION_ON;
      U     "DB_GRP_82".PP40.SM.MotorOn;
      U(    ;
      UN    "DB_POWER_SAVING_MODE2".GENERAL.SM.PR_MODE_2_ON;
      U(    ;
      U     "82CLM82_R.H>R.H_SETPOINT";
      U(    ;
      O     "COMM_0";
      O     "COMM_1";
      )     ;
      O     "82CLT81_T>T_SETPOINT";
      )     ;
      O     ;
      U     "DB_POWER_SAVING_MODE2".GENERAL.SM.PR_MODE_2_ON;
      U(    ;
      O     "DB_POWER_SAVING_MODE2".MODE.PR_ARU_COOLING;
      O     "DB_POWER_SAVING_MODE2".MODE.PR_ARU_DEHUMIDIFYING;
      )     ;
      )     ;
      U(    ;
      O     "DBI_PID_ARU_PR".QLMNDN;
      ON    "DBI_PID_ARU_PR".QLMNDN;
      )     ;
      UN    "DB_Gest_ES".FLAG._081;
      =     #AutoOn;
      U     L      6.0;
      U(    ;
      UN    "DB_POWER_SAVING_MODE2".GENERAL.SM.PR_MODE_2_ON;
      U     "DBI_PID_ARU_PR".QLMNUP;
      UN    "DBI_PID_ARU_PR".QLMNUP;
      O     ;
      U     "DB_POWER_SAVING_MODE2".GENERAL.SM.PR_MODE_2_ON;
      U(    ;
      U(    ;
      O     "DB_POWER_SAVING_MODE2".MODE.PR_ARU_COOLING;
      O     "DB_POWER_SAVING_MODE2".MODE.PR_ARU_DEHUMIDIFYING;
      )     ;
      U     "DBI_PID_ARU_PR".QLMNUP;
      O     ;
      UN    "DB_POWER_SAVING_MODE2".MODE.PR_ARU_COOLING;
      UN    "DB_POWER_SAVING_MODE2".MODE.PR_ARU_DEHUMIDIFYING;
      )     ;
      O     ;
      U     "DB_PROG".PRIMER.SM.ARU_REGULATION_ON;
      UN    "DB_GRP_82".PID_ARU.SM.CTRL_On;
      O     ;
      U     "PR_STOP_PROD_FANS";
      U     "T_ARU_STOP_DELAY";
      ON    "DB_PROG".PRIMER.SM.ARU_REGULATION_ON;
      O     "DB_GRP_82".FAN91.SM.GeneralError;
      O     "DB_GRP_82".FAN92.SM.GeneralError;
      O     "DB_GRP_80".FAN61.SM.GeneralError;
      O     "DB_GRP_80".FAN81.SM.GeneralError;
      O     "DB_GRP_82".FAN91_PRESSURE.FM.L01_MinErr;
      O     "DB_GRP_82".FAN92_PRESSURE.FM.L01_MinErr;
      O     "DB_GRP_82".FAN91_PRESSURE.FM.Alarm;
      O     "DB_GRP_82".FAN92_PRESSURE.FM.Alarm;
      O     "DB_Gest_ES".FLAG._081;
      )     ;
      =     #AutoOff;
NETWORK
TITLE =FIRE ALARM CLOSE
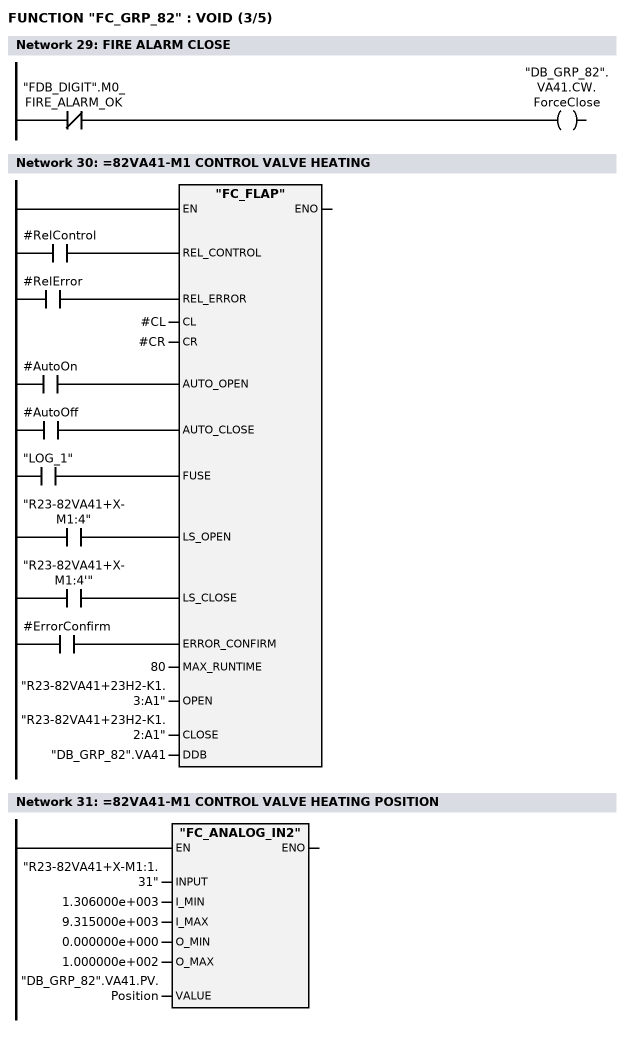
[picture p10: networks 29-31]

      UN    "FDB_DIGIT".M0_FIRE_ALARM_OK;
      =     "DB_GRP_82".VA41.CW.ForceClose;
NETWORK
TITLE ==82VA41-M1 CONTROL VALVE HEATING

      U     #RelControl;
      =     L      6.0;
      BLD   103;
      U     #RelError;
      =     L      6.1;
      BLD   103;
      U     #AutoOn;
      =     L      6.2;
      BLD   103;
      U     #AutoOff;
      =     L      6.3;
      BLD   103;
      U     "LOG_1";
      =     L      6.4;
      BLD   103;
      U     "R23-82VA41+X-M1:4";
      =     L      6.5;
      BLD   103;
      U     "R23-82VA41+X-M1:4'";
      =     L      6.6;
      BLD   103;
      U     #ErrorConfirm;
      =     L      6.7;
      BLD   103;
      CALL "FC_FLAP" (
           REL_CONTROL              := L      6.0,
           REL_ERROR                := L      6.1,
           CL                       := #CL,
           CR                       := #CR,
           AUTO_OPEN                := L      6.2,
           AUTO_CLOSE               := L      6.3,
           FUSE                     := L      6.4,
           LS_OPEN                  := L      6.5,
           LS_CLOSE                 := L      6.6,
           ERROR_CONFIRM            := L      6.7,
           MAX_RUNTIME              := 80,
           OPEN                     := "R23-82VA41+23H2-K1.3:A1",
           CLOSE                    := "R23-82VA41+23H2-K1.2:A1",
           DDB                      := "DB_GRP_82".VA41);
      NOP   0;
NETWORK
TITLE ==82VA41-M1 CONTROL VALVE HEATING POSITION

      CALL "FC_ANALOG_IN2" (
           INPUT                    := "R23-82VA41+X-M1:1.31",
           I_MIN                    := 1.306000e+003,
           I_MAX                    := 9.315000e+003,
           O_MIN                    := 0.000000e+000,
           O_MAX                    := 1.000000e+002,
           VALUE                    := "DB_GRP_82".VA41.PV.Position);
      NOP   0;
NETWORK
TITLE ==82FTR80-B33 FILTER PRESSURE MONITORING
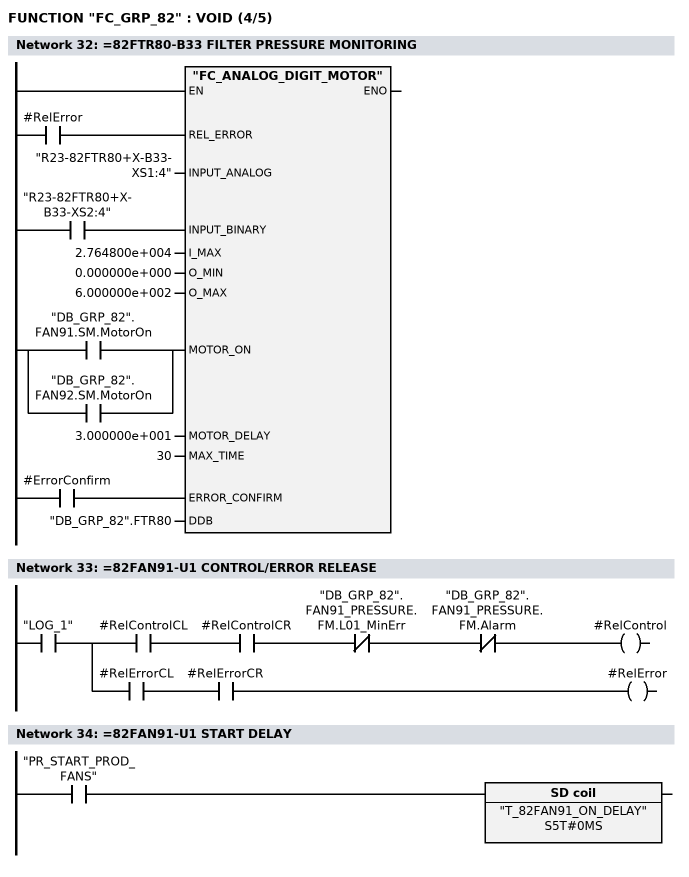
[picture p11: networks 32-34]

      U     #RelError;
      =     L      6.0;
      BLD   103;
      U     "R23-82FTR80+X-B33-XS2:4";
      =     L      6.1;
      BLD   103;
      U(    ;
      O     "DB_GRP_82".FAN91.SM.MotorOn;
      O     "DB_GRP_82".FAN92.SM.MotorOn;
      )     ;
      =     L      6.2;
      BLD   103;
      U     #ErrorConfirm;
      =     L      6.3;
      BLD   103;
      CALL "FC_ANALOG_DIGIT_MOTOR" (
           REL_ERROR                := L      6.0,
           INPUT_ANALOG             := "R23-82FTR80+X-B33-XS1:4",
           INPUT_BINARY             := L      6.1,
           I_MAX                    := 2.764800e+004,
           O_MIN                    := 0.000000e+000,
           O_MAX                    := 6.000000e+002,
           MOTOR_ON                 := L      6.2,
           MOTOR_DELAY              := 3.000000e+001,
           MAX_TIME                 := 30,
           ERROR_CONFIRM            := L      6.3,
           DDB                      := "DB_GRP_82".FTR80);
      NOP   0;
NETWORK
TITLE ==82FAN91-U1 CONTROL/ERROR RELEASE

      U     "LOG_1";
      =     L      6.0;
      U     L      6.0;
      U     #RelControlCL;
      U     #RelControlCR;
      UN    "DB_GRP_82".FAN91_PRESSURE.FM.L01_MinErr;
      UN    "DB_GRP_82".FAN91_PRESSURE.FM.Alarm;
      =     #RelControl;
      U     L      6.0;
      U     #RelErrorCL;
      U     #RelErrorCR;
      =     #RelError;
NETWORK
TITLE ==82FAN91-U1 START DELAY

      U     "PR_START_PROD_FANS";
      L     S5T#0MS;
      SE    "T_82FAN91_ON_DELAY";
      NOP   0;
      NOP   0;
      NOP   0;
      NOP   0;
NETWORK
TITLE ==82FAN91-U1 CONTROL SIGNALS
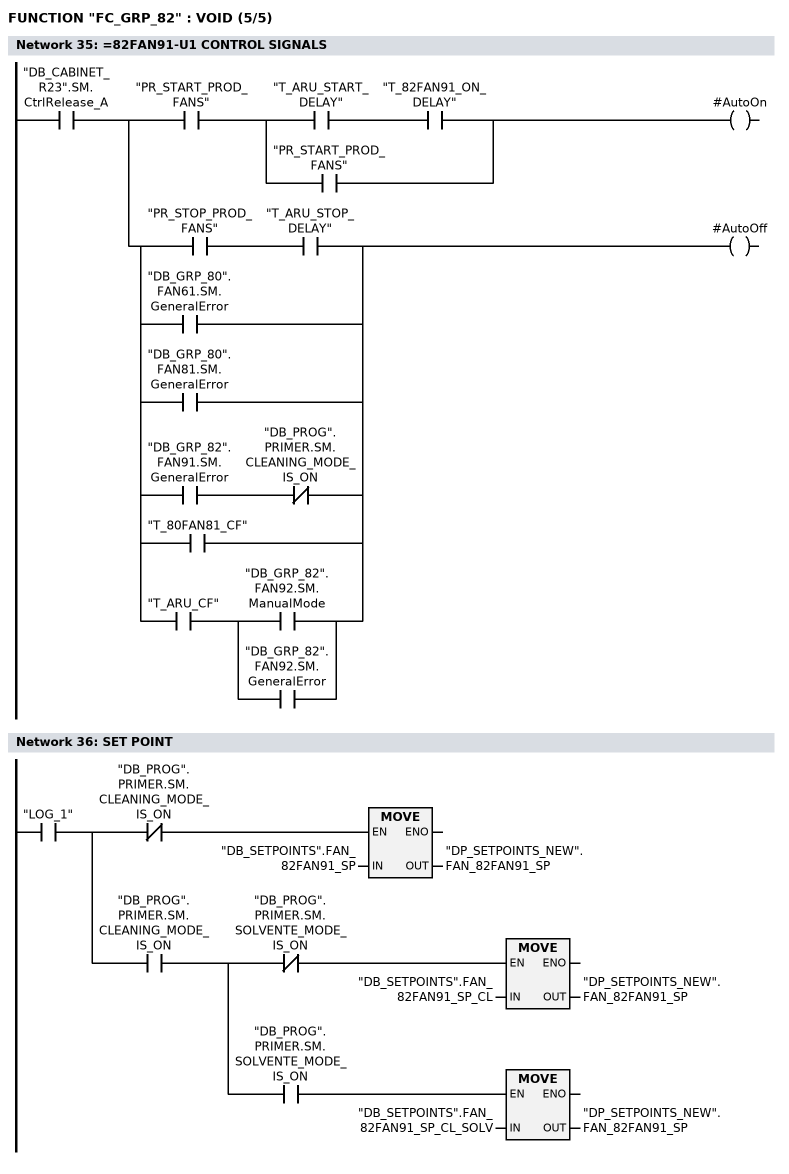
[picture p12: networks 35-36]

      U     "DB_CABINET_R23".SM.CtrlRelease_A;
      =     L      6.0;
      U     L      6.0;
      U     "PR_START_PROD_FANS";
      U(    ;
      U     "T_ARU_START_DELAY";
      U     "T_82FAN91_ON_DELAY";
      O     "PR_START_PROD_FANS";
      )     ;
      =     #AutoOn;
      U     L      6.0;
      U(    ;
      U     "PR_STOP_PROD_FANS";
      U     "T_ARU_STOP_DELAY";
      O     "DB_GRP_80".FAN61.SM.GeneralError;
      O     "DB_GRP_80".FAN81.SM.GeneralError;
      O     ;
      U     "DB_GRP_82".FAN91.SM.GeneralError;
      UN    "DB_PROG".PRIMER.SM.CLEANING_MODE_IS_ON;
      O     "T_80FAN81_CF";
      O     ;
      U     "T_ARU_CF";
      U(    ;
      O     "DB_GRP_82".FAN92.SM.ManualMode;
      O     "DB_GRP_82".FAN92.SM.GeneralError;
      )     ;
      )     ;
      =     #AutoOff;
NETWORK
TITLE =SET POINT

      U     "LOG_1";
      =     L      6.0;
      U     L      6.0;
      UN    "DB_PROG".PRIMER.SM.CLEANING_MODE_IS_ON;
      SPBNB _006;
      L     "DB_SETPOINTS".FAN_82FAN91_SP;
      T     "DP_SETPOINTS_NEW".FAN_82FAN91_SP;
_006: NOP   0;
      U     L      6.0;
      U     "DB_PROG".PRIMER.SM.CLEANING_MODE_IS_ON;
      =     L      6.1;
      U     L      6.1;
      UN    "DB_PROG".PRIMER.SM.SOLVENTE_MODE_IS_ON;
      SPBNB _007;
      L     "DB_SETPOINTS".FAN_82FAN91_SP_CL;
      T     "DP_SETPOINTS_NEW".FAN_82FAN91_SP;
_007: NOP   0;
      U     L      6.1;
      U     "DB_PROG".PRIMER.SM.SOLVENTE_MODE_IS_ON;
      SPBNB _008;
      L     "DB_SETPOINTS".FAN_82FAN91_SP_CL_SOLV;
      T     "DP_SETPOINTS_NEW".FAN_82FAN91_SP;
_008: NOP   0;
NETWORK
TITLE =SALVA E RIPRISTINA SETPOIN PRESSIONE 82FAN91

      U     "LOG_1";
      =     L      6.0;
      U     L      6.0;
      U     "DB_PROG".PRIMER.SM.CLEANING_MODE_IS_ON;
      FP    "M230.0";
      =     L      6.1;
      U     L      6.1;
      SPBNB _009;
      L     "DB_GRP_82".FAN91_PRESSURE.PV.Limit_04;
      T     "DP_SETPOINTS_NEW".FAN_82FAN91_PRESS_LIM_04;
_009: NOP   0;
      U     L      6.1;
      SPBNB _00a;
      L     "DB_GRP_82".FAN91_PRESSURE.PV.Limit_03;
      T     "DP_SETPOINTS_NEW".FAN_82FAN91_PRESS_LIM_03;
_00a: NOP   0;
      U     L      6.1;
      SPBNB _00b;
      L     "DB_GRP_82".FAN91_PRESSURE.PV.Limit_02;
      T     "DP_SETPOINTS_NEW".FAN_82FAN91_PRESS_LIM_02;
_00b: NOP   0;
      U     L      6.1;
      SPBNB _00c;
      L     "DB_GRP_82".FAN91_PRESSURE.PV.Limit_01;
      T     "DP_SETPOINTS_NEW".FAN_82FAN91_PRESS_LIM_01;
_00c: NOP   0;
      U     L      6.0;
      UN    "DB_PROG".PRIMER.SM.CLEANING_MODE_IS_ON;
      FP    "M230.1";
      =     L      6.1;
      U     L      6.1;
      SPBNB _00d;
      L     "DP_SETPOINTS_NEW".FAN_82FAN91_PRESS_LIM_04;
      T     "DB_GRP_82".FAN91_PRESSURE.PV.Limit_04;
_00d: NOP   0;
      U     L      6.1;
      SPBNB _00e;
      L     "DP_SETPOINTS_NEW".FAN_82FAN91_PRESS_LIM_03;
      T     "DB_GRP_82".FAN91_PRESSURE.PV.Limit_03;
_00e: NOP   0;
      U     L      6.1;
      SPBNB _00f;
      L     "DP_SETPOINTS_NEW".FAN_82FAN91_PRESS_LIM_02;
      T     "DB_GRP_82".FAN91_PRESSURE.PV.Limit_02;
_00f: NOP   0;
      U     L      6.1;
      SPBNB _010;
      L     "DP_SETPOINTS_NEW".FAN_82FAN91_PRESS_LIM_01;
      T     "DB_GRP_82".FAN91_PRESSURE.PV.Limit_01;
_010: NOP   0;
NETWORK
TITLE =SETPOIN MOD PULIZIA PRESSIONE 82FAN91

      U(    ;
      U     "LOG_1";
      U     "DB_PROG".PRIMER.SM.CLEANING_MODE_IS_ON;
      L     S5T#1S;
      SE    "T41";
      NOP   0;
      NOP   0;
      NOP   0;
      U     "T41";
      )     ;
      FP    "M230.2";
      =     L      6.0;
      U     L      6.0;
      SPBNB _011;
      L     1.100000e+003;
      T     "DB_GRP_82".FAN91_PRESSURE.PV.Limit_04;
_011: NOP   0;
      U     L      6.0;
      SPBNB _012;
      L     1.000000e+003;
      T     "DB_GRP_82".FAN91_PRESSURE.PV.Limit_03;
_012: NOP   0;
      U     L      6.0;
      SPBNB _013;
      L     4.000000e+002;
      T     "DB_GRP_82".FAN91_PRESSURE.PV.Limit_02;
_013: NOP   0;
      U     L      6.0;
      SPBNB _014;
      L     3.000000e+002;
      T     "DB_GRP_82".FAN91_PRESSURE.PV.Limit_01;
_014: NOP   0;
NETWORK
TITLE ==82FAN91-U1 REDUCE SPEED
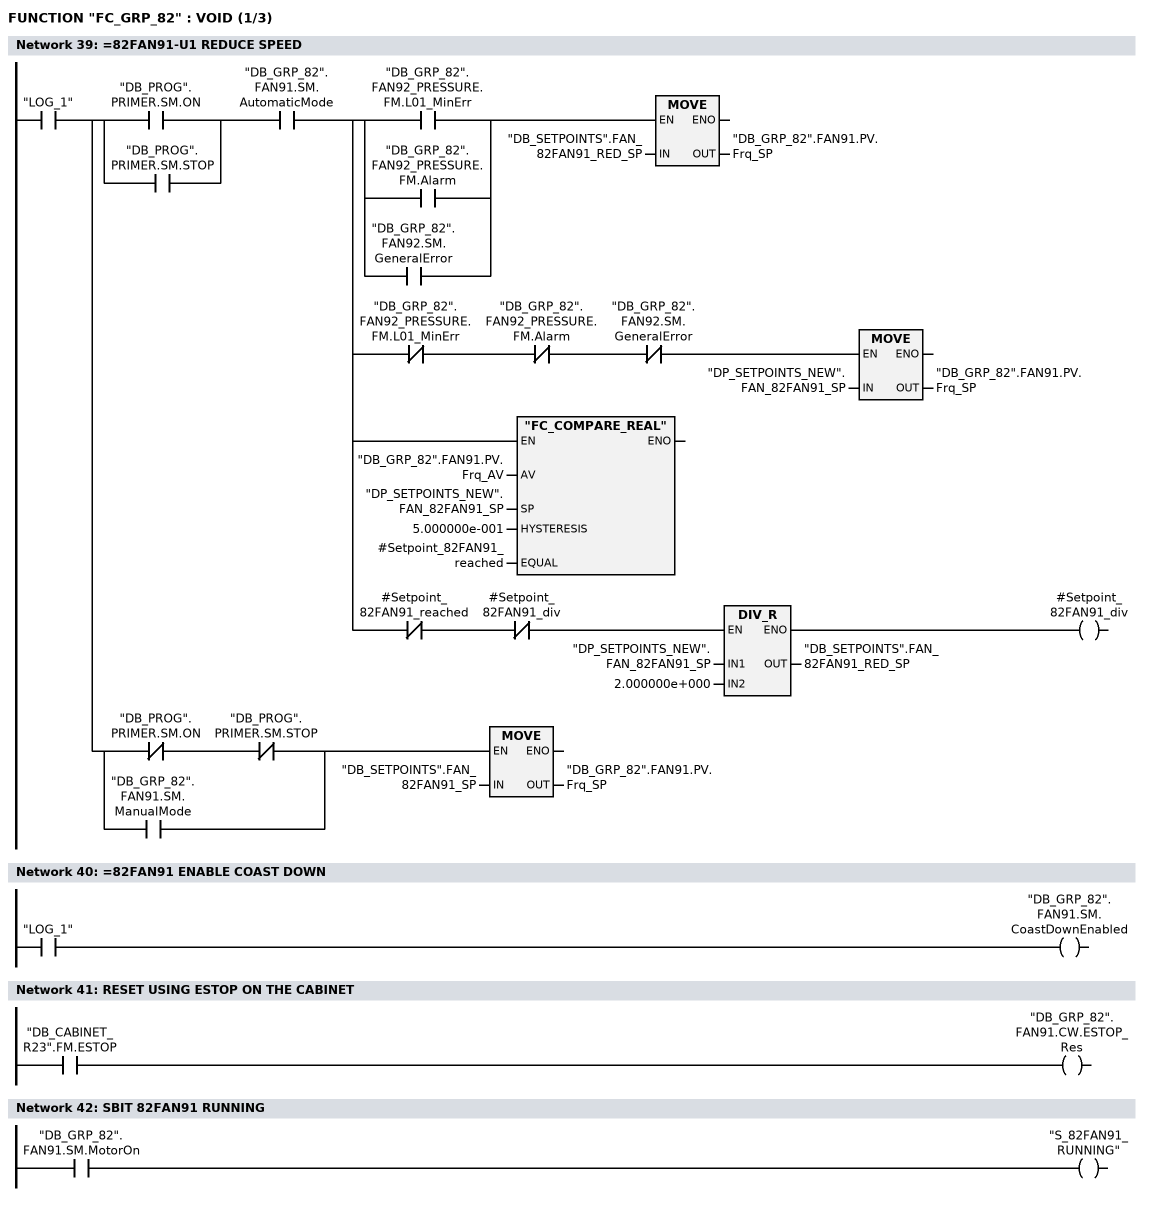
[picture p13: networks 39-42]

      U     "LOG_1";
      =     L      6.0;
      U     L      6.0;
      U(    ;
      O     "DB_PROG".PRIMER.SM.ON;
      O     "DB_PROG".PRIMER.SM.STOP;
      )     ;
      U     "DB_GRP_82".FAN91.SM.AutomaticMode;
      =     L      6.1;
      U     L      6.1;
      U(    ;
      O     "DB_GRP_82".FAN92_PRESSURE.FM.L01_MinErr;
      O     "DB_GRP_82".FAN92_PRESSURE.FM.Alarm;
      O     "DB_GRP_82".FAN92.SM.GeneralError;
      )     ;
      SPBNB _015;
      L     "DB_SETPOINTS".FAN_82FAN91_RED_SP;
      T     "DB_GRP_82".FAN91.PV.Frq_SP;
_015: NOP   0;
      U     L      6.1;
      UN    "DB_GRP_82".FAN92_PRESSURE.FM.L01_MinErr;
      UN    "DB_GRP_82".FAN92_PRESSURE.FM.Alarm;
      UN    "DB_GRP_82".FAN92.SM.GeneralError;
      SPBNB _016;
      L     "DP_SETPOINTS_NEW".FAN_82FAN91_SP;
      T     "DB_GRP_82".FAN91.PV.Frq_SP;
_016: NOP   0;
      U     L      6.1;
      SPBNB _017;
      CALL "FC_COMPARE_REAL" (
           AV                       := "DB_GRP_82".FAN91.PV.Frq_AV,
           SP                       := "DP_SETPOINTS_NEW".FAN_82FAN91_SP,
           HYSTERESIS               := 5.000000e-001,
           EQUAL                    := #Setpoint_82FAN91_reached);
_017: NOP   0;
      U     L      6.1;
      UN    #Setpoint_82FAN91_reached;
      UN    #Setpoint_82FAN91_div;
      SPBNB _018;
      L     "DP_SETPOINTS_NEW".FAN_82FAN91_SP;
      L     2.000000e+000;
      /R    ;
      T     "DB_SETPOINTS".FAN_82FAN91_RED_SP;
      UN    OV;
      SAVE  ;
      CLR   ;
_018: U     BIE;
      =     #Setpoint_82FAN91_div;
      U     L      6.0;
      U(    ;
      UN    "DB_PROG".PRIMER.SM.ON;
      UN    "DB_PROG".PRIMER.SM.STOP;
      O     "DB_GRP_82".FAN91.SM.ManualMode;
      )     ;
      SPBNB _019;
      L     "DB_SETPOINTS".FAN_82FAN91_SP;
      T     "DB_GRP_82".FAN91.PV.Frq_SP;
_019: NOP   0;
NETWORK
TITLE ==82FAN91 ENABLE COAST DOWN

      U     "LOG_1";
      =     "DB_GRP_82".FAN91.SM.CoastDownEnabled;
NETWORK
TITLE =RESET USING ESTOP ON THE CABINET

      U     "DB_CABINET_R23".FM.ESTOP;
      =     "DB_GRP_82".FAN91.CW.ESTOP_Res;


NETWORK
TITLE =SBIT 82FAN91 RUNNING

      U     "DB_GRP_82".FAN91.SM.MotorOn;
      =     "S_82FAN91_RUNNING";
NETWORK
TITLE ==82FAN91-U1 EXHAUST AIR FAN
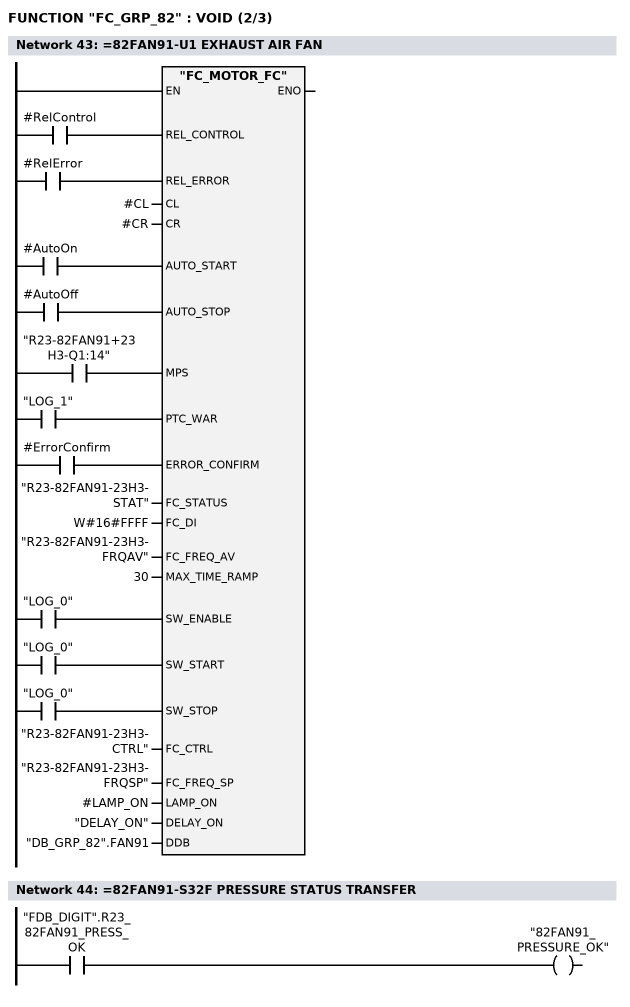
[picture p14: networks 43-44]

      U     #RelControl;
      =     L      6.0;
      BLD   103;
      U     #RelError;
      =     L      6.1;
      BLD   103;
      U     #AutoOn;
      =     L      6.2;
      BLD   103;
      U     #AutoOff;
      =     L      6.3;
      BLD   103;
      U     "R23-82FAN91+23H3-Q1:14";
      =     L      6.4;
      BLD   103;
      U     "LOG_1";
      =     L      6.5;
      BLD   103;
      U     #ErrorConfirm;
      =     L      6.6;
      BLD   103;
      U     "LOG_0";
      =     L      6.7;
      BLD   103;
      U     "LOG_0";
      =     L      7.0;
      BLD   103;
      U     "LOG_0";
      =     L      7.1;
      BLD   103;
      CALL "FC_MOTOR_FC" (
           REL_CONTROL              := L      6.0,
           REL_ERROR                := L      6.1,
           CL                       := #CL,
           CR                       := #CR,
           AUTO_START               := L      6.2,
           AUTO_STOP                := L      6.3,
           MPS                      := L      6.4,
           PTC_WAR                  := L      6.5,
           ERROR_CONFIRM            := L      6.6,
           FC_STATUS                := "R23-82FAN91-23H3-STAT",
           FC_DI                    := W#16#FFFF,
           FC_FREQ_AV               := "R23-82FAN91-23H3-FRQAV",
           MAX_TIME_RAMP            := 30,
           SW_ENABLE                := L      6.7,
           SW_START                 := L      7.0,
           SW_STOP                  := L      7.1,
           FC_CTRL                  := "R23-82FAN91-23H3-CTRL",
           FC_FREQ_SP               := "R23-82FAN91-23H3-FRQSP",
           LAMP_ON                  := #LAMP_ON,
           DELAY_ON                 := "DELAY_ON",
           DDB                      := "DB_GRP_82".FAN91);
      NOP   0;
NETWORK
TITLE ==82FAN91-S32F PRESSURE STATUS TRANSFER

      U     "FDB_DIGIT".R23_82FAN91_PRESS_OK;
      =     "82FAN91_PRESSURE_OK";
NETWORK
TITLE ==82FAN91-S32F PRESSURE MONITORING
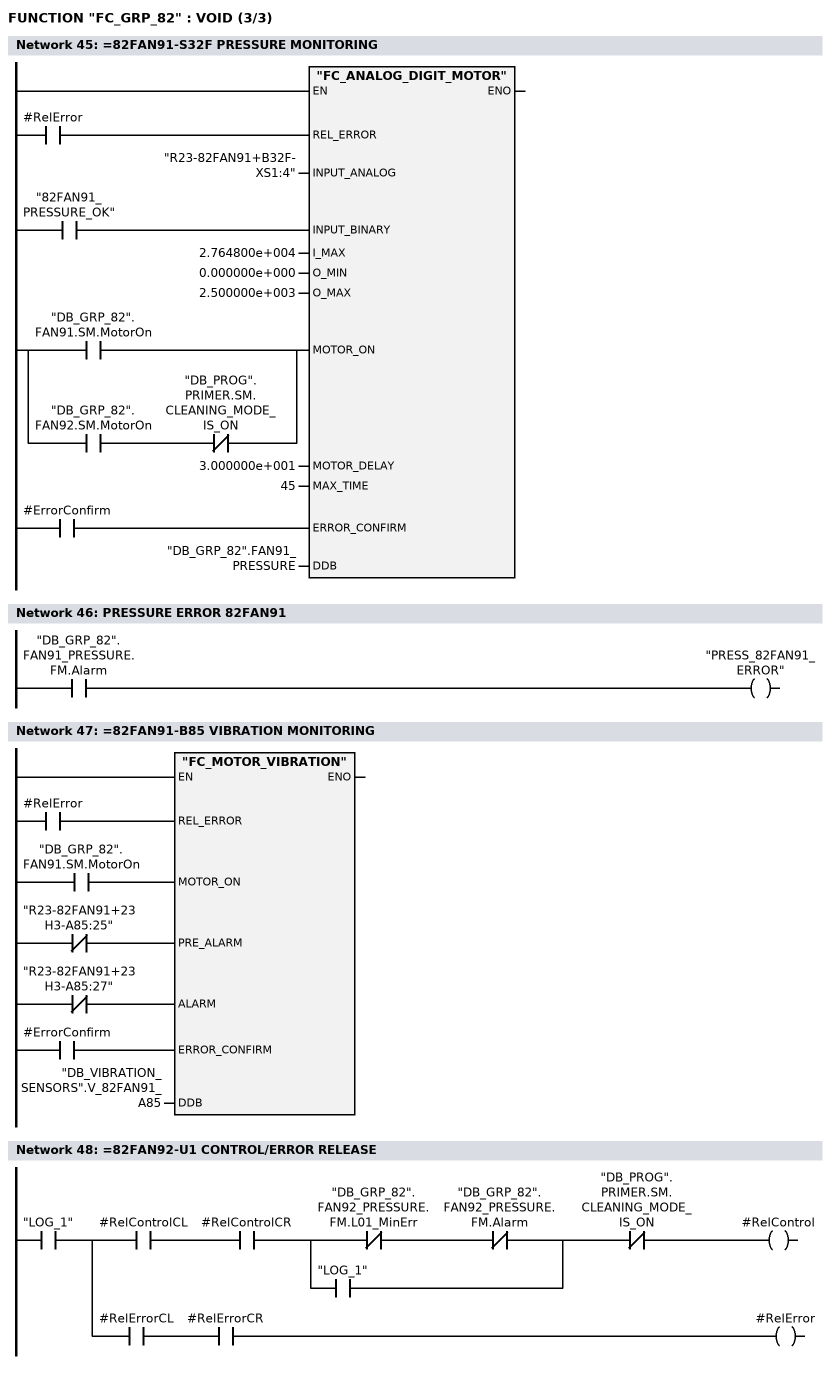
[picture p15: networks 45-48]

      U     #RelError;
      =     L      6.0;
      BLD   103;
      U     "82FAN91_PRESSURE_OK";
      =     L      6.1;
      BLD   103;
      U(    ;
      O     "DB_GRP_82".FAN91.SM.MotorOn;
      O     ;
      U     "DB_GRP_82".FAN92.SM.MotorOn;
      UN    "DB_PROG".PRIMER.SM.CLEANING_MODE_IS_ON;
      )     ;
      =     L      6.2;
      BLD   103;
      U     #ErrorConfirm;
      =     L      6.3;
      BLD   103;
      CALL "FC_ANALOG_DIGIT_MOTOR" (
           REL_ERROR                := L      6.0,
           INPUT_ANALOG             := "R23-82FAN91+B32F-XS1:4",
           INPUT_BINARY             := L      6.1,
           I_MAX                    := 2.764800e+004,
           O_MIN                    := 0.000000e+000,
           O_MAX                    := 2.500000e+003,
           MOTOR_ON                 := L      6.2,
           MOTOR_DELAY              := 3.000000e+001,
           MAX_TIME                 := 45,
           ERROR_CONFIRM            := L      6.3,
           DDB                      := "DB_GRP_82".FAN91_PRESSURE);
      NOP   0;
NETWORK
TITLE =PRESSURE ERROR 82FAN91

      U     "DB_GRP_82".FAN91_PRESSURE.FM.Alarm;
      =     "PRESS_82FAN91_ERROR";
NETWORK
TITLE ==82FAN91-B85 VIBRATION MONITORING

      U     #RelError;
      =     L      6.0;
      BLD   103;
      U     "DB_GRP_82".FAN91.SM.MotorOn;
      =     L      6.1;
      BLD   103;
      UN    "R23-82FAN91+23H3-A85:25";
      =     L      6.2;
      BLD   103;
      UN    "R23-82FAN91+23H3-A85:27";
      =     L      6.3;
      BLD   103;
      U     #ErrorConfirm;
      =     L      6.4;
      BLD   103;
      CALL "FC_MOTOR_VIBRATION" (
           REL_ERROR                := L      6.0,
           MOTOR_ON                 := L      6.1,
           PRE_ALARM                := L      6.2,
           ALARM                    := L      6.3,
           ERROR_CONFIRM            := L      6.4,
           DDB                      := "DB_VIBRATION_SENSORS".V_82FAN91_A85);
      NOP   0;
NETWORK
TITLE ==82FAN92-U1 CONTROL/ERROR RELEASE

      U     "LOG_1";
      =     L      6.0;
      U     L      6.0;
      U     #RelControlCL;
      U     #RelControlCR;
      U(    ;
      UN    "DB_GRP_82".FAN92_PRESSURE.FM.L01_MinErr;
      UN    "DB_GRP_82".FAN92_PRESSURE.FM.Alarm;
      O     "LOG_1";
      )     ;
      UN    "DB_PROG".PRIMER.SM.CLEANING_MODE_IS_ON;
      =     #RelControl;
      U     L      6.0;
      U     #RelErrorCL;
      U     #RelErrorCR;
      =     #RelError;
NETWORK
TITLE ==82FAN92-U1 CONTROL SIGNALS

      U     "DB_CABINET_R23".SM.CtrlRelease_A;
      =     L      6.0;
      U     L      6.0;
      U     "PR_START_PROD_FANS";
      =     L      6.1;
      U     L      6.1;
      U     "T_ARU_START_DELAY";
      UN    "DB_PROG".PRIMER.SM.CLEANING_MODE_IS_ON;
      L     S5T#10S;
      SE    "T_82FAN92_ON_DELAY";
      NOP   0;
      NOP   0;
      NOP   0;
      U     "T_82FAN92_ON_DELAY";
      =     #AutoOn;
      U     L      6.1;
      U     "PR_START_PROD_FANS";
      =     #AutoOn;
      U     L      6.0;
      U(    ;
      U     "PR_STOP_PROD_FANS";
      U     "T_ARU_STOP_DELAY";
      O     "DB_PROG".PRIMER.SM.CLEANING_MODE_IS_ON;
      O     "DB_GRP_80".FAN61.SM.GeneralError;
      O     "DB_GRP_80".FAN81.SM.GeneralError;
      O     "DB_GRP_82".FAN92.SM.GeneralError;
      O     "T_80FAN81_CF";
      O     ;
      U     "T_ARU_CF";
      U(    ;
      O     "DB_GRP_82".FAN91.SM.ManualMode;
      O     "DB_GRP_82".FAN91.SM.GeneralError;
      )     ;
      )     ;
      =     #AutoOff;
NETWORK
TITLE ==82FAN92-U1 REDUCE SPEED
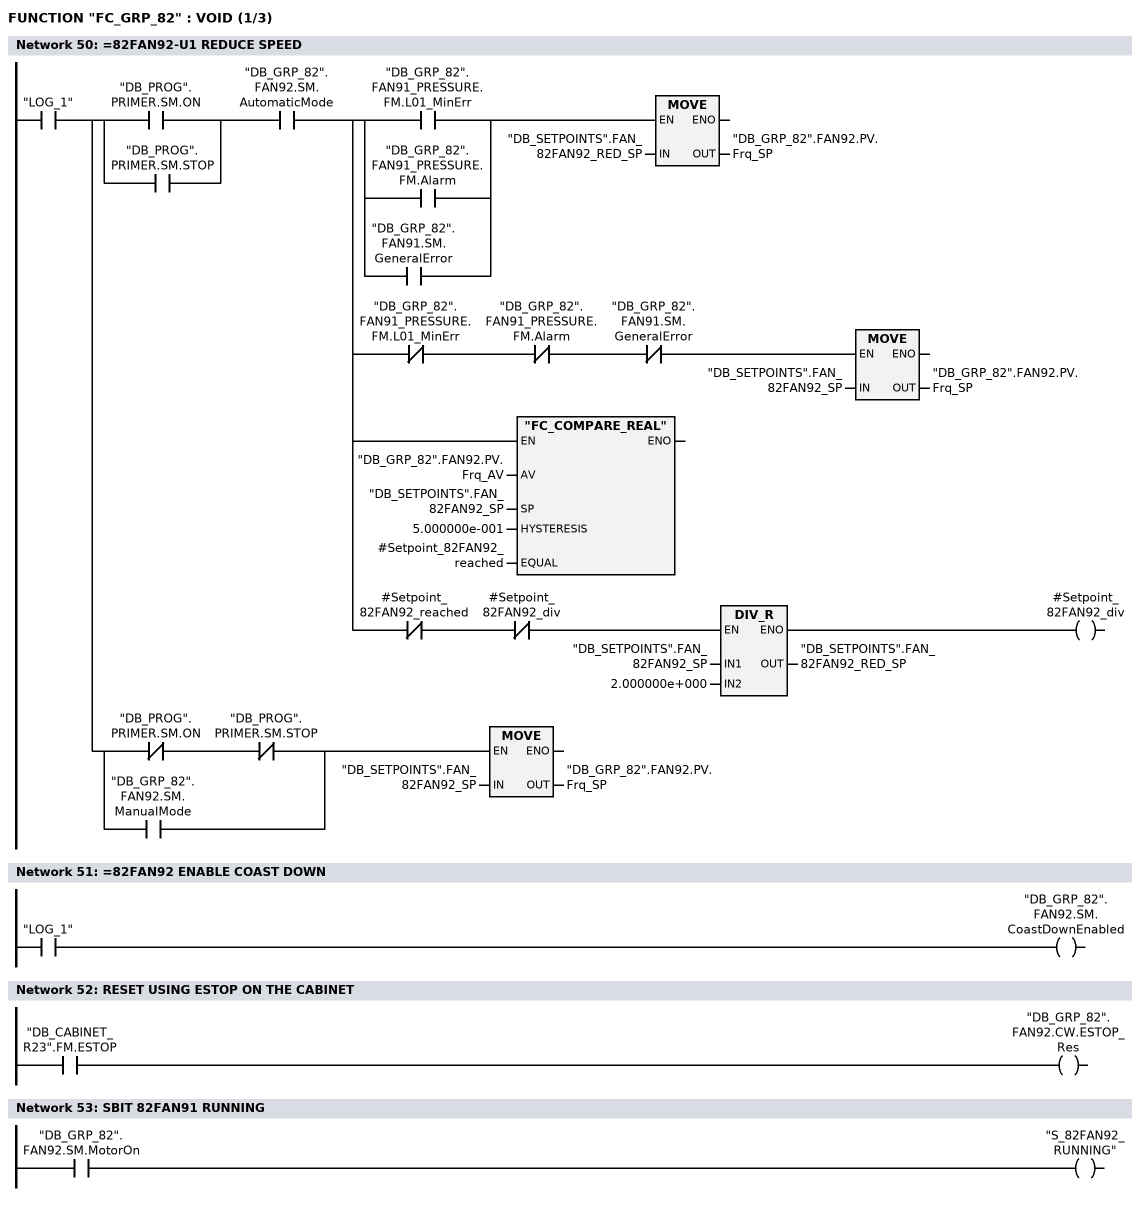
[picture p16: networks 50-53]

      U     "LOG_1";
      =     L      6.0;
      U     L      6.0;
      U(    ;
      O     "DB_PROG".PRIMER.SM.ON;
      O     "DB_PROG".PRIMER.SM.STOP;
      )     ;
      U     "DB_GRP_82".FAN92.SM.AutomaticMode;
      =     L      6.1;
      U     L      6.1;
      U(    ;
      O     "DB_GRP_82".FAN91_PRESSURE.FM.L01_MinErr;
      O     "DB_GRP_82".FAN91_PRESSURE.FM.Alarm;
      O     "DB_GRP_82".FAN91.SM.GeneralError;
      )     ;
      SPBNB _01a;
      L     "DB_SETPOINTS".FAN_82FAN92_RED_SP;
      T     "DB_GRP_82".FAN92.PV.Frq_SP;
_01a: NOP   0;
      U     L      6.1;
      UN    "DB_GRP_82".FAN91_PRESSURE.FM.L01_MinErr;
      UN    "DB_GRP_82".FAN91_PRESSURE.FM.Alarm;
      UN    "DB_GRP_82".FAN91.SM.GeneralError;
      SPBNB _01b;
      L     "DB_SETPOINTS".FAN_82FAN92_SP;
      T     "DB_GRP_82".FAN92.PV.Frq_SP;
_01b: NOP   0;
      U     L      6.1;
      SPBNB _01c;
      CALL "FC_COMPARE_REAL" (
           AV                       := "DB_GRP_82".FAN92.PV.Frq_AV,
           SP                       := "DB_SETPOINTS".FAN_82FAN92_SP,
           HYSTERESIS               := 5.000000e-001,
           EQUAL                    := #Setpoint_82FAN92_reached);
_01c: NOP   0;
      U     L      6.1;
      UN    #Setpoint_82FAN92_reached;
      UN    #Setpoint_82FAN92_div;
      SPBNB _01d;
      L     "DB_SETPOINTS".FAN_82FAN92_SP;
      L     2.000000e+000;
      /R    ;
      T     "DB_SETPOINTS".FAN_82FAN92_RED_SP;
      UN    OV;
      SAVE  ;
      CLR   ;
_01d: U     BIE;
      =     #Setpoint_82FAN92_div;
      U     L      6.0;
      U(    ;
      UN    "DB_PROG".PRIMER.SM.ON;
      UN    "DB_PROG".PRIMER.SM.STOP;
      O     "DB_GRP_82".FAN92.SM.ManualMode;
      )     ;
      SPBNB _01e;
      L     "DB_SETPOINTS".FAN_82FAN92_SP;
      T     "DB_GRP_82".FAN92.PV.Frq_SP;
_01e: NOP   0;
NETWORK
TITLE ==82FAN92 ENABLE COAST DOWN

      U     "LOG_1";
      =     "DB_GRP_82".FAN92.SM.CoastDownEnabled;
NETWORK
TITLE =RESET USING ESTOP ON THE CABINET

      U     "DB_CABINET_R23".FM.ESTOP;
      =     "DB_GRP_82".FAN92.CW.ESTOP_Res;
NETWORK
TITLE =SBIT 82FAN91 RUNNING

      U     "DB_GRP_82".FAN92.SM.MotorOn;
      =     "S_82FAN92_RUNNING";
NETWORK
TITLE ==82FAN92-U1 EXHAUST AIR FAN
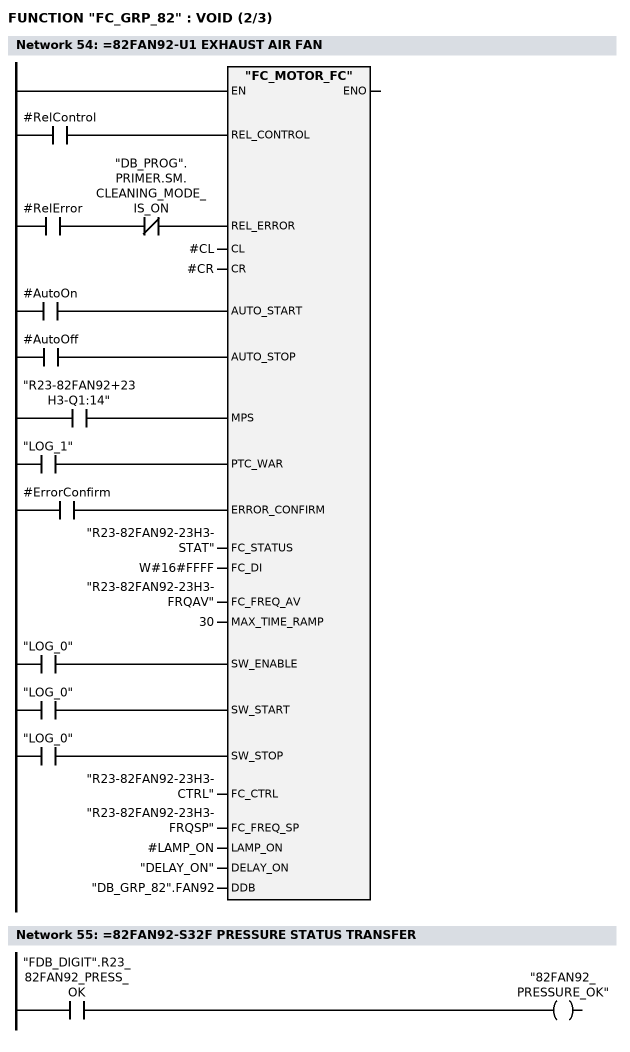
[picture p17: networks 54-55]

      U     #RelControl;
      =     L      6.0;
      BLD   103;
      U     #RelError;
      UN    "DB_PROG".PRIMER.SM.CLEANING_MODE_IS_ON;
      =     L      6.1;
      BLD   103;
      U     #AutoOn;
      =     L      6.2;
      BLD   103;
      U     #AutoOff;
      =     L      6.3;
      BLD   103;
      U     "R23-82FAN92+23H3-Q1:14";
      =     L      6.4;
      BLD   103;
      U     "LOG_1";
      =     L      6.5;
      BLD   103;
      U     #ErrorConfirm;
      =     L      6.6;
      BLD   103;
      U     "LOG_0";
      =     L      6.7;
      BLD   103;
      U     "LOG_0";
      =     L      7.0;
      BLD   103;
      U     "LOG_0";
      =     L      7.1;
      BLD   103;
      CALL "FC_MOTOR_FC" (
           REL_CONTROL              := L      6.0,
           REL_ERROR                := L      6.1,
           CL                       := #CL,
           CR                       := #CR,
           AUTO_START               := L      6.2,
           AUTO_STOP                := L      6.3,
           MPS                      := L      6.4,
           PTC_WAR                  := L      6.5,
           ERROR_CONFIRM            := L      6.6,
           FC_STATUS                := "R23-82FAN92-23H3-STAT",
           FC_DI                    := W#16#FFFF,
           FC_FREQ_AV               := "R23-82FAN92-23H3-FRQAV",
           MAX_TIME_RAMP            := 30,
           SW_ENABLE                := L      6.7,
           SW_START                 := L      7.0,
           SW_STOP                  := L      7.1,
           FC_CTRL                  := "R23-82FAN92-23H3-CTRL",
           FC_FREQ_SP               := "R23-82FAN92-23H3-FRQSP",
           LAMP_ON                  := #LAMP_ON,
           DELAY_ON                 := "DELAY_ON",
           DDB                      := "DB_GRP_82".FAN92);
      NOP   0;
NETWORK
TITLE ==82FAN92-S32F PRESSURE STATUS TRANSFER

      U     "FDB_DIGIT".R23_82FAN92_PRESS_OK;
      =     "82FAN92_PRESSURE_OK";
NETWORK
TITLE ==82FAN92-S32F PRESSURE MONITORING
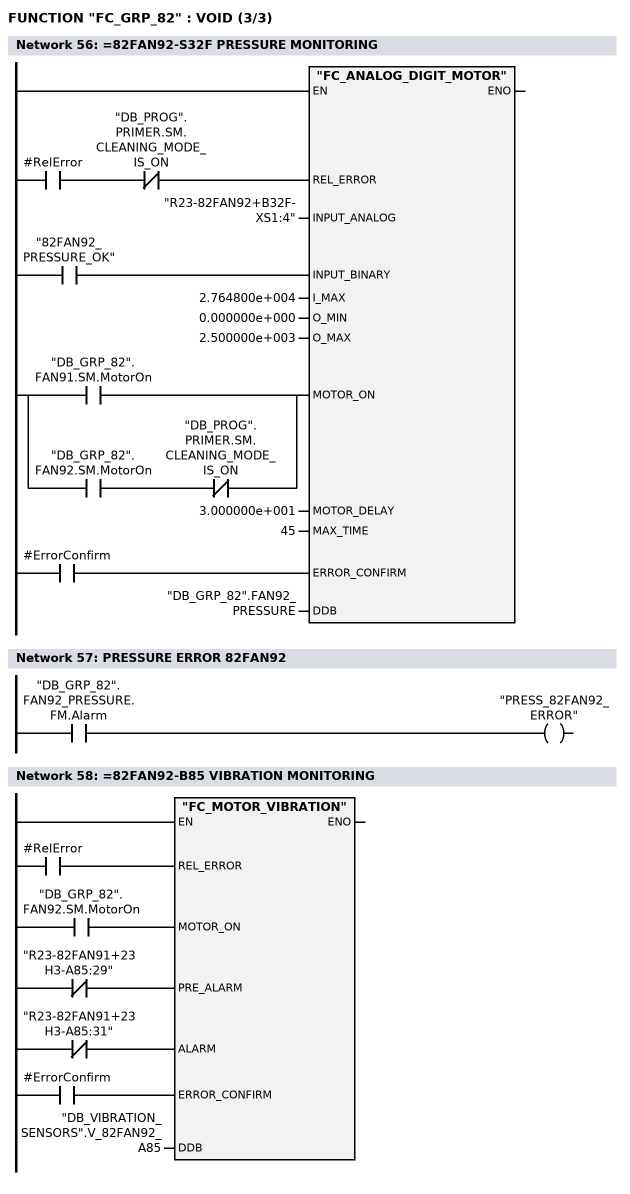
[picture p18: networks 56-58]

      U     #RelError;
      UN    "DB_PROG".PRIMER.SM.CLEANING_MODE_IS_ON;
      =     L      6.0;
      BLD   103;
      U     "82FAN92_PRESSURE_OK";
      =     L      6.1;
      BLD   103;
      U(    ;
      O     "DB_GRP_82".FAN91.SM.MotorOn;
      O     ;
      U     "DB_GRP_82".FAN92.SM.MotorOn;
      UN    "DB_PROG".PRIMER.SM.CLEANING_MODE_IS_ON;
      )     ;
      =     L      6.2;
      BLD   103;
      U     #ErrorConfirm;
      =     L      6.3;
      BLD   103;
      CALL "FC_ANALOG_DIGIT_MOTOR" (
           REL_ERROR                := L      6.0,
           INPUT_ANALOG             := "R23-82FAN92+B32F-XS1:4",
           INPUT_BINARY             := L      6.1,
           I_MAX                    := 2.764800e+004,
           O_MIN                    := 0.000000e+000,
           O_MAX                    := 2.500000e+003,
           MOTOR_ON                 := L      6.2,
           MOTOR_DELAY              := 3.000000e+001,
           MAX_TIME                 := 45,
           ERROR_CONFIRM            := L      6.3,
           DDB                      := "DB_GRP_82".FAN92_PRESSURE);
      NOP   0;
NETWORK
TITLE =PRESSURE ERROR 82FAN92

      U     "DB_GRP_82".FAN92_PRESSURE.FM.Alarm;
      =     "PRESS_82FAN92_ERROR";
NETWORK
TITLE ==82FAN92-B85 VIBRATION MONITORING

      U     #RelError;
      =     L      6.0;
      BLD   103;
      U     "DB_GRP_82".FAN92.SM.MotorOn;
      =     L      6.1;
      BLD   103;
      UN    "R23-82FAN91+23H3-A85:29";
      =     L      6.2;
      BLD   103;
      UN    "R23-82FAN91+23H3-A85:31";
      =     L      6.3;
      BLD   103;
      U     #ErrorConfirm;
      =     L      6.4;
      BLD   103;
      CALL "FC_MOTOR_VIBRATION" (
           REL_ERROR                := L      6.0,
           MOTOR_ON                 := L      6.1,
           PRE_ALARM                := L      6.2,
           ALARM                    := L      6.3,
           ERROR_CONFIRM            := L      6.4,
           DDB                      := "DB_VIBRATION_SENSORS".V_82FAN92_A85);
      NOP   0;
NETWORK
TITLE =END



END_FUNCTION

